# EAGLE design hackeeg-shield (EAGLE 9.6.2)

## Sheet 1 of 4: ADS1299 and power supplies
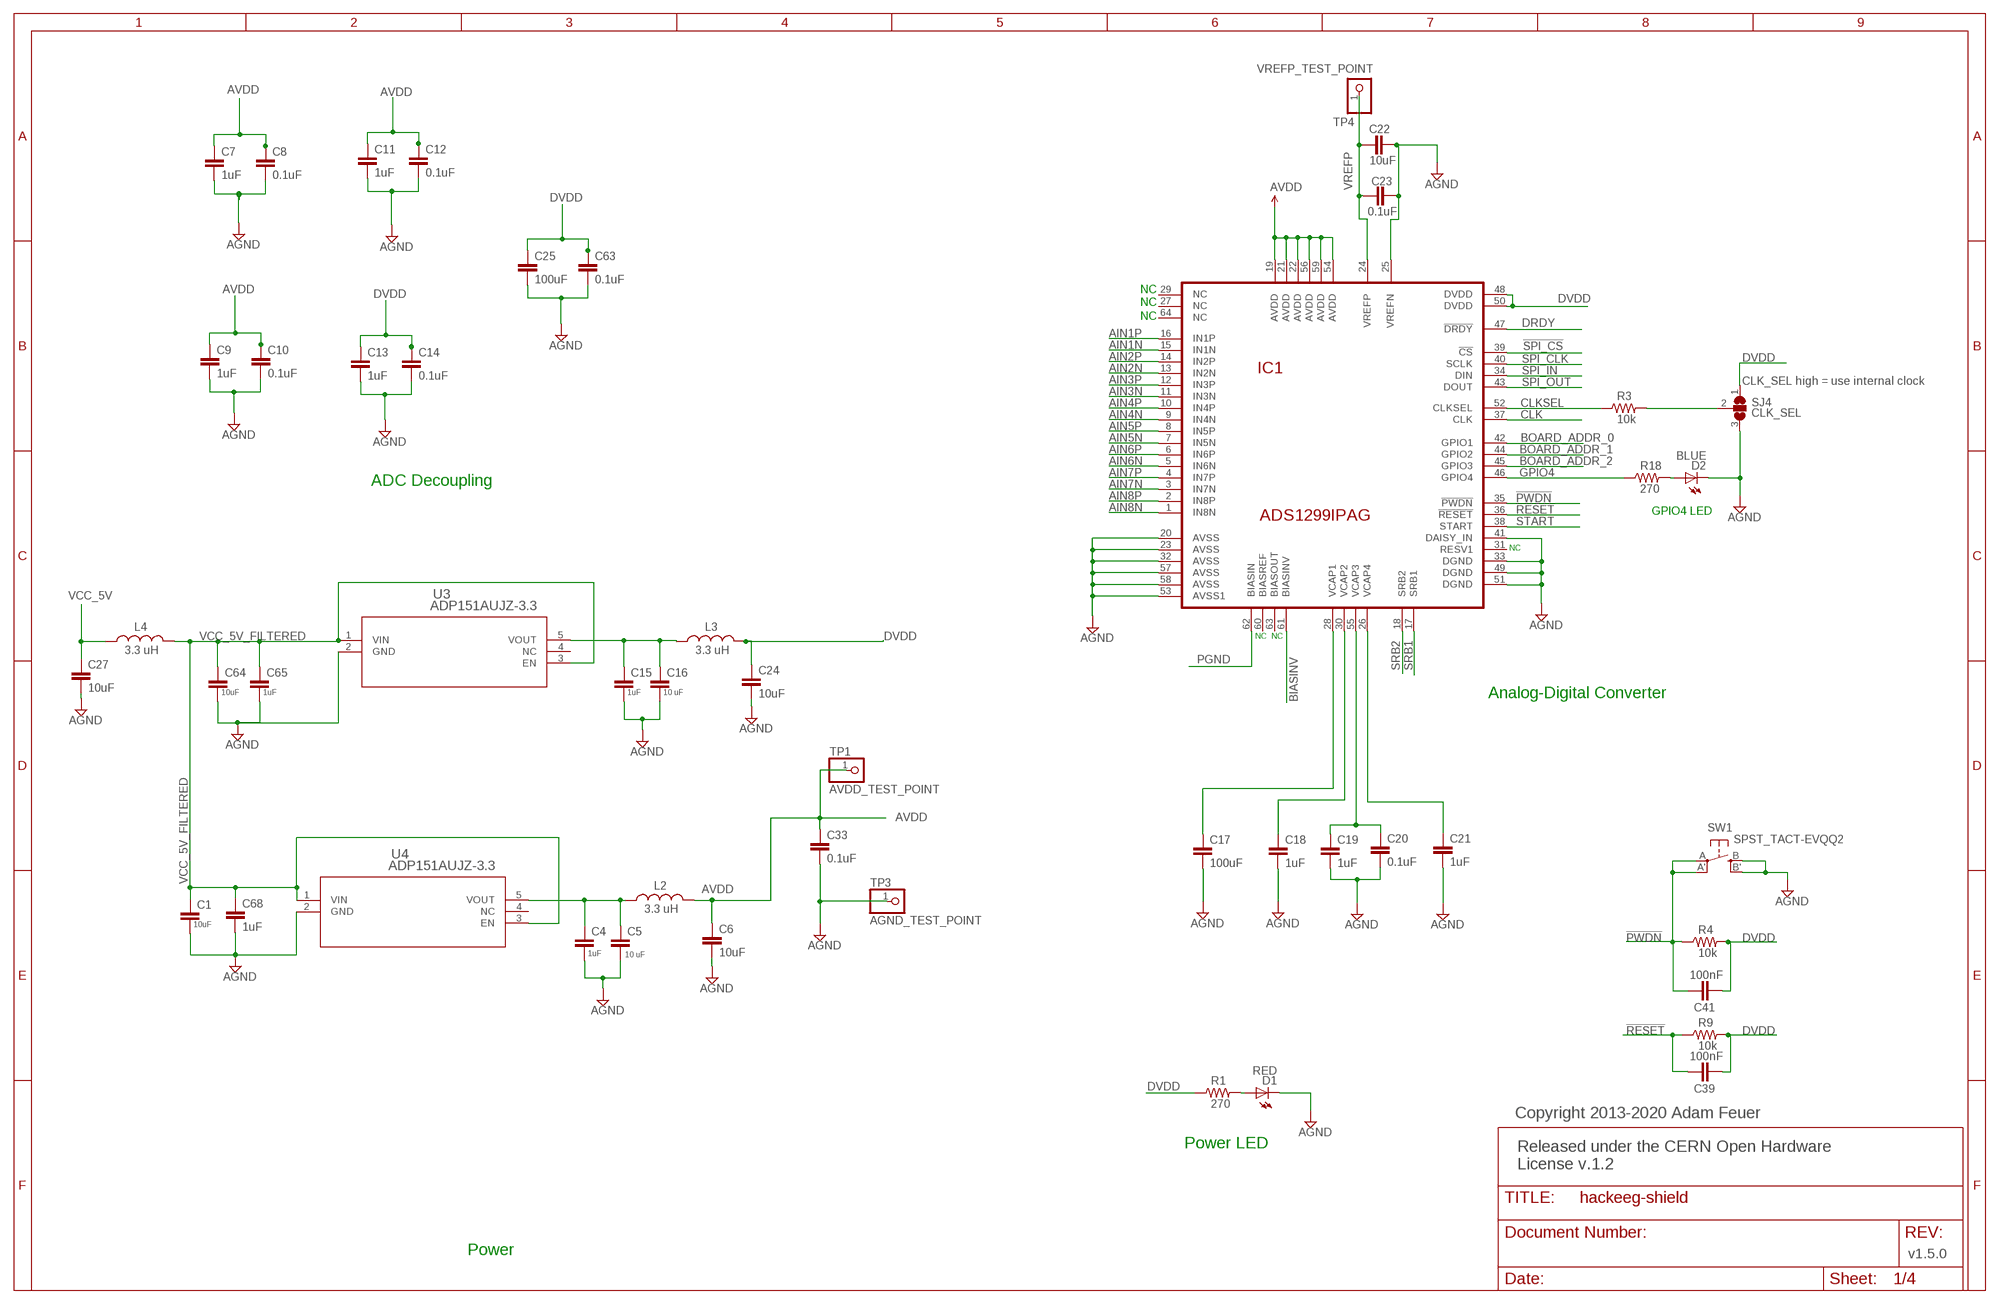
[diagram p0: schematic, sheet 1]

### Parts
C1  10uF  CAP0603-CAP  [0603-CAP]
C4  1uF  CAP0603-CAP  [0603-CAP]
C5  10 uF  CAP0603-CAP  [0603-CAP]
C6  10uF  CAP0603-CAP  [0603-CAP]
C7  1uF  CAP0603-CAP  [0603-CAP]
C8  0.1uF  CAP0603-CAP  [0603-CAP]
C9  1uF  CAP0603-CAP  [0603-CAP]
C10  0.1uF  CAP0603-CAP  [0603-CAP]
C11  1uF  CAP0603-CAP  [0603-CAP]
C12  0.1uF  CAP0603-CAP  [0603-CAP]
C13  1uF  CAP0603-CAP  [0603-CAP]
C14  0.1uF  CAP0603-CAP  [0603-CAP]
C15  1uF  CAP0603-CAP  [0603-CAP]
C16  10 uF  CAP0603-CAP  [0603-CAP]
C17  100uF  CAP1210  [1210]
C18  1uF  CAP0603-CAP  [0603-CAP]
C19  1uF  CAP0603-CAP  [0603-CAP]
C20  0.1uF  CAP0603-CAP  [0603-CAP]
C21  1uF  CAP0603-CAP  [0603-CAP]
C22  10uF  CAP0603-CAP  [0603-CAP]
C23  0.1uF  CAP0603-CAP  [0603-CAP]
C24  10uF  CAP0603-CAP  [0603-CAP]
C25  100uF  CAP1210  [1210]
C27  10uF  CAP0603-CAP  [0603-CAP]
C33  0.1uF  CAP0603-CAP  [0603-CAP]
C39  100nF  CAP0603-CAP  [0603-CAP]
C41  100nF  CAP0603-CAP  [0603-CAP]
C63  0.1uF  CAP0603-CAP  [0603-CAP]
C64  10uF  CAP0603-CAP  [0603-CAP]
C65  1uF  CAP0603-CAP  [0603-CAP]
C68  1uF  CAP0603-CAP  [0603-CAP]
D1  RED  LED-RED1206  [LED-1206]
D2  BLUE  LED-WHITE  [LED-1206]
IC1  ADS1299IPAG  ADS1299*PAG*  [TQFP64]
L2  3.3 uH  INDUCTOR0805  [0805]
L3  3.3 uH  INDUCTOR0805  [0805]
L4  3.3 uH  INDUCTOR0805  [0805]
R1  270  RESISTOR0603-RES  [0603-RES]
R3  10k  RESISTOR0603-RES  [0603-RES]
R4  10k  RESISTOR0603-RES  [0603-RES]
R9  10k  RESISTOR0603-RES  [0603-RES]
R18  270  RESISTOR0603-RES  [0603-RES]
SJ4  CLK_SEL  SJ2W  [SJ_2]
SW1  SPST_TACT-EVQQ2  [EVQ-Q2]
TP1  AVDD_TEST_POINT  PINHD-1X1  [1X01]
TP3  AGND_TEST_POINT  PINHD-1X1  [1X01]
TP4  VREFP_TEST_POINT  PINHD-1X1  [1X01]
U3  ADP151AUJZ-3.3  [UJ_5_ADI]
U4  ADP151AUJZ-3.3  [UJ_5_ADI]

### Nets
!PWDN: C41.1 IC1.35(!PWDN) R4.1 SW1.A'(P1) SW1.A(P)
!RESET: C39.1 IC1.36(!RESET) R9.1
!SPI_CS: IC1.39(!CS) ; also sheet 3
AGND: C1.2 C4.2 C5.2 C6.2 C7.2 C8.2 C9.2 C10.2 C11.2 C12.2 C13.2 C14.2 C15.2 C16.2 C17.2 C18.2 C19.2 C20.2 C21.2 C22.2 C23.2 C24.2 C25.2 C27.2 C33.2 C63.2 C64.2 C65.2 C68.2 D1.C D2.C IC1.20(AVSS) IC1.23(AVSS) IC1.25(VREFN) IC1.32(AVSS) IC1.33(DGND) IC1.41(DAISY_IN) IC1.49(DGND) IC1.51(DGND) IC1.53(AVSS1) IC1.57(AVSS) IC1.58(AVSS) SJ4.3 SW1.B'(S1) SW1.B(S) TP3.1 U3.2(GND) U4.2(GND) ; also sheet 2,3
AIN1N: IC1.15(IN1N) ; also sheet 2
AIN1P: IC1.16(IN1P) ; also sheet 2
AIN2N: IC1.13(IN2N) ; also sheet 2
AIN2P: IC1.14(IN2P) ; also sheet 2
AIN3N: IC1.11(IN3N) ; also sheet 2
AIN3P: IC1.12(IN3P) ; also sheet 2
AIN4N: IC1.9(IN4N) ; also sheet 2
AIN4P: IC1.10(IN4P) ; also sheet 2
AIN5N: IC1.7(IN5N) ; also sheet 2
AIN5P: IC1.8(IN5P) ; also sheet 2
AIN6N: IC1.5(IN6N) ; also sheet 2
AIN6P: IC1.6(IN6P) ; also sheet 2
AIN7N: IC1.3(IN7N) ; also sheet 2
AIN7P: IC1.4(IN7P) ; also sheet 2
AIN8N: IC1.1(IN8N) ; also sheet 2
AIN8P: IC1.2(IN8P) ; also sheet 2
AVDD: C6.1 C7.1 C8.1 C9.1 C10.1 C11.1 C12.1 C33.1 IC1.19(AVDD) IC1.21(AVDD) IC1.22(AVDD) IC1.54(AVDD) IC1.56(AVDD) IC1.59(AVDD) L2.2 TP1.1 ; also sheet 2
BIASINV: IC1.61(BIASINV) ; also sheet 2
BOARD_ADDR_0: IC1.42(GPIO1)
BOARD_ADDR_1: IC1.44(GPIO2)
BOARD_ADDR_2: IC1.45(GPIO3)
CLK: IC1.37(CLK) ; also sheet 3
CLKSEL: IC1.52(CLKSEL) R3.1
DRDY: IC1.47(!DRDY) ; also sheet 3
DVDD: C13.1 C14.1 C24.1 C25.1 C39.2 C41.2 C63.1 IC1.48(DVDD) IC1.50(DVDD) L3.2 R1.1 R4.2 R9.2 SJ4.1 ; also sheet 3
GPIO4: IC1.46(GPIO4) R18.1
N$1: C4.1 C5.1 L2.1 U4.5(VOUT)
N$2: C15.1 C16.1 L3.1 U3.5(VOUT)
N$3: C17.1 IC1.28(VCAP1)
N$4: C18.1 IC1.30(VCAP2)
N$5: C19.1 C20.1 IC1.55(VCAP3)
N$8: C21.1 IC1.26(VCAP4)
N$14: D2.A R18.2
N$19: D1.A R1.2
N$20: R3.2 SJ4.2
PGND: IC1.62(BIASIN) ; also sheet 2
SPI_CLK: IC1.40(SCLK) ; also sheet 3
SPI_IN: IC1.34(DIN) ; also sheet 3
SPI_OUT: IC1.43(DOUT) ; also sheet 3
SRB1: IC1.17(SRB1) ; also sheet 2
SRB2: IC1.18(SRB2) ; also sheet 3
START: IC1.38(START) ; also sheet 3
VCC_5V: C27.1 L4.1 ; also sheet 3
VCC_5V_FILTERED: C1.1 C64.1 C65.1 C68.1 L4.2 U3.1(VIN) U3.3(EN) U4.1(VIN) U4.3(EN)
VREFP: C22.1 C23.1 IC1.24(VREFP) TP4.1
Unconnected: IC1.27(NC) IC1.29(NC) IC1.31(RESV1) IC1.60(BIASREF) IC1.63(BIASOUT) IC1.64(NC) U3.4(NC) U4.4(NC)

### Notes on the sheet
- NC
- NC
- NC
- CLK_SEL high = use internal clock
- ADC Decoupling
- GPIO4 LED
- NC
- NC | NC
- Analog-Digital Converter
- Copyright 2013-2020 Adam Feuer
- Power LED
- Released under the CERN Open Hardware 
  License v.1.2
- Power | v1.5.0

## Sheet 2 of 4: Input filtering and electrode connector
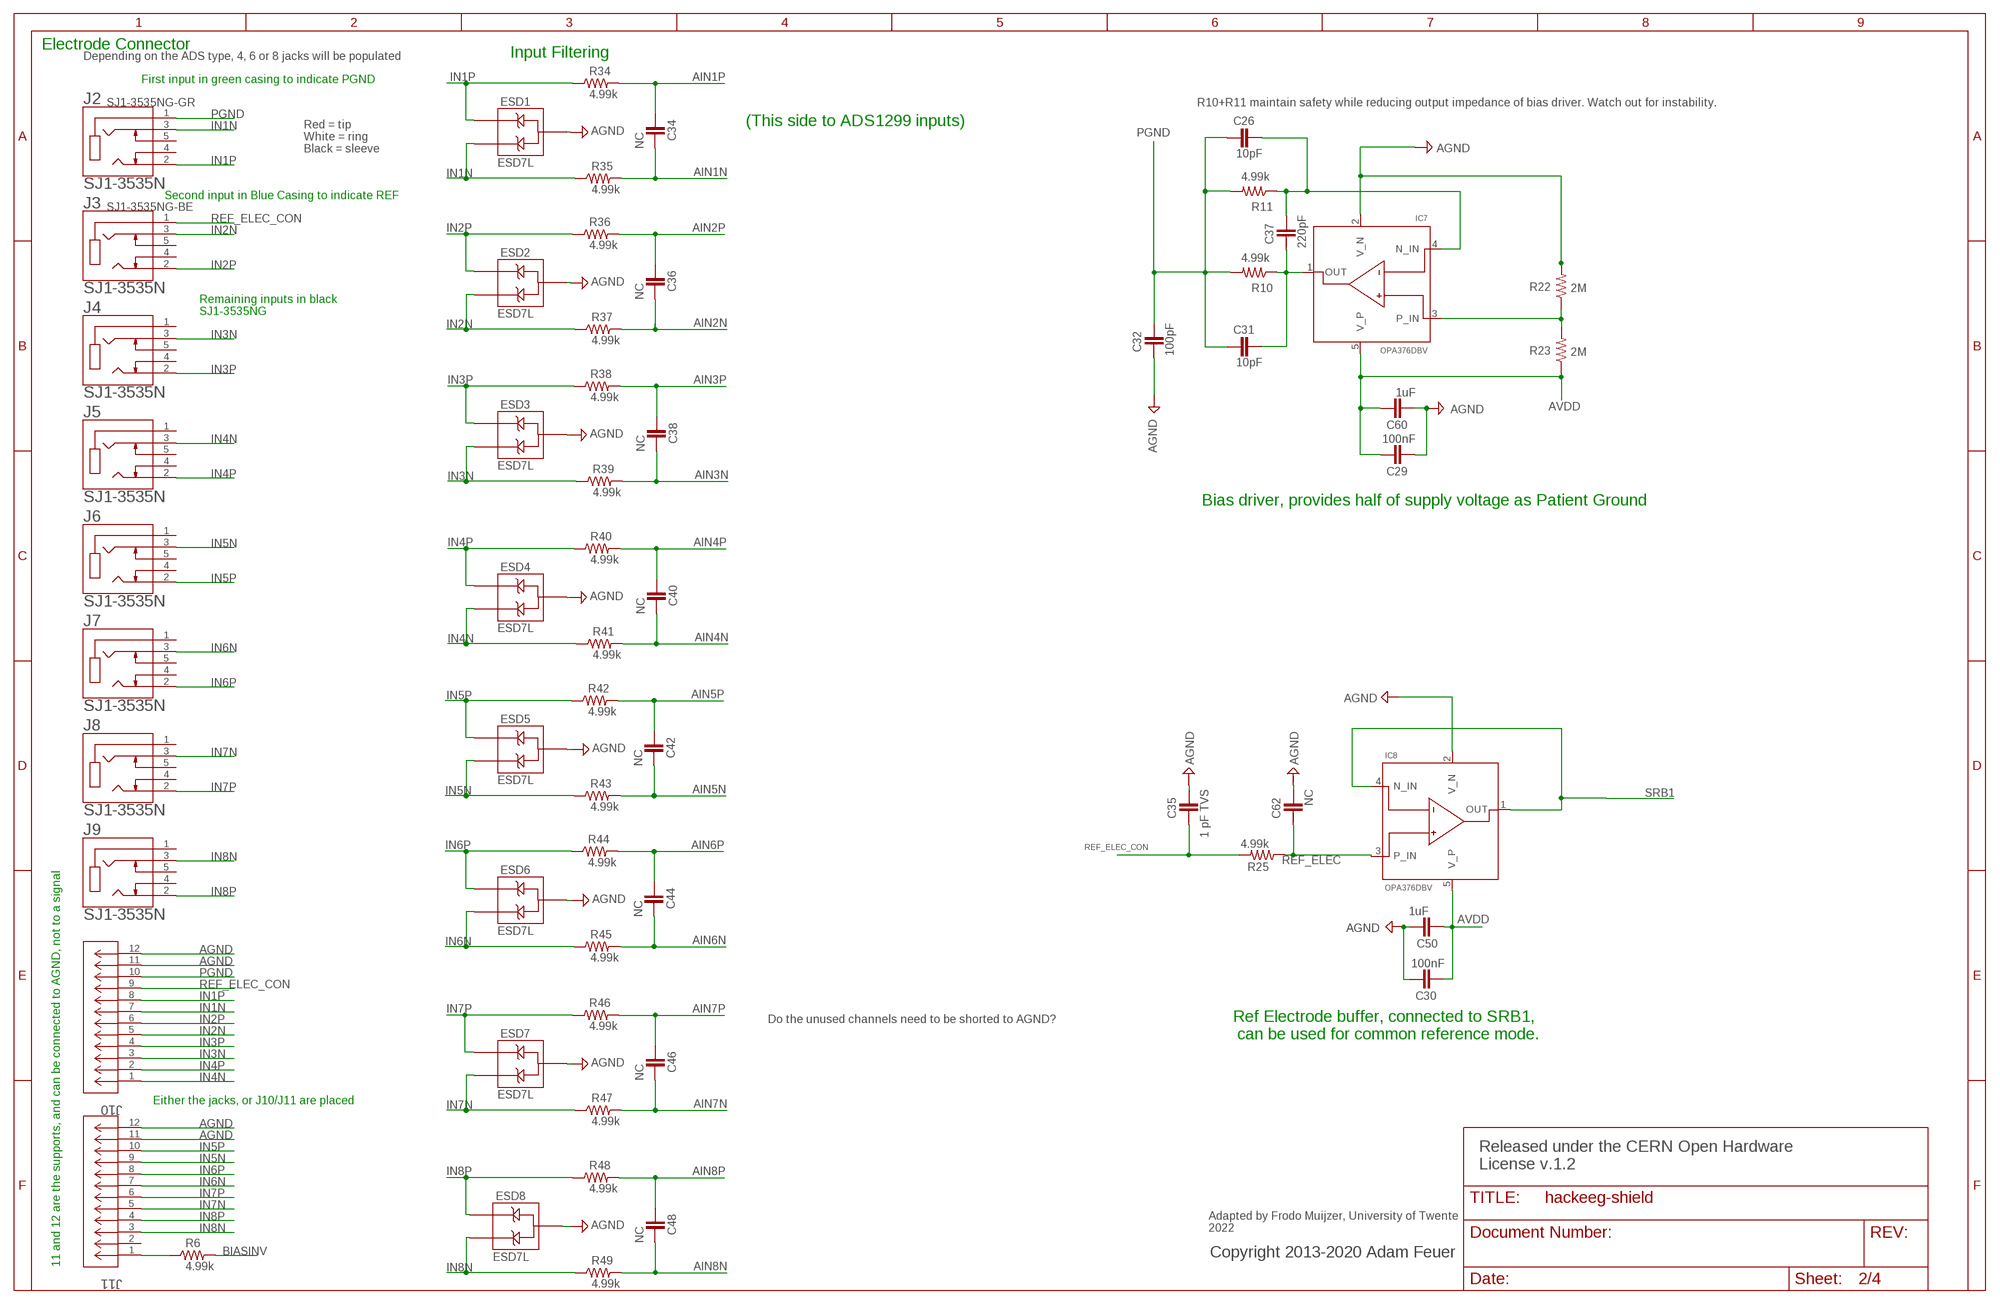
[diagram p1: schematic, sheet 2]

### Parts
C26  10pF  CAP0603-CAP  [0603-CAP]
C29  100nF  CAP0603-CAP  [0603-CAP]
C30  100nF  CAP0603-CAP  [0603-CAP]
C31  10pF  CAP0603-CAP  [0603-CAP]
C32  100pF  CAP0603-CAP  [0603-CAP]
C34  NC  CAP0603-CAP  [0603-CAP]
C35  1 pF TVS  CAP0603-CAP  [0603-CAP]
C36  NC  CAP0603-CAP  [0603-CAP]
C37  220pF  CAP0603-CAP  [0603-CAP]
C38  NC  CAP0603-CAP  [0603-CAP]
C40  NC  CAP0603-CAP  [0603-CAP]
C42  NC  CAP0603-CAP  [0603-CAP]
C44  NC  CAP0603-CAP  [0603-CAP]
C46  NC  CAP0603-CAP  [0603-CAP]
C48  NC  CAP0603-CAP  [0603-CAP]
C50  1uF  CAP0603-CAP  [0603-CAP]
C60  1uF  CAP0603-CAP  [0603-CAP]
C62  NC  CAP0603-CAP  [0603-CAP]
ESD1  ESD7L  [SOT-723]
ESD2  ESD7L  [SOT-723]
ESD3  ESD7L  [SOT-723]
ESD4  ESD7L  [SOT-723]
ESD5  ESD7L  [SOT-723]
ESD6  ESD7L  [SOT-723]
ESD7  ESD7L  [SOT-723]
ESD8  ESD7L  [SOT-723]
IC7  OPA376DBV  [SOT23-5]
IC8  OPA376DBV  [SOT23-5]
J2  SJ1-3535N  [CUI_SJ1-3535N]
J3  SJ1-3535N  [CUI_SJ1-3535N]
J4  SJ1-3535N  [CUI_SJ1-3535N]
J5  SJ1-3535N  [CUI_SJ1-3535N]
J6  SJ1-3535N  [CUI_SJ1-3535N]
J7  SJ1-3535N  [CUI_SJ1-3535N]
J8  SJ1-3535N  [CUI_SJ1-3535N]
J9  SJ1-3535N  [CUI_SJ1-3535N]
J10  533981071  [CON_533981071]
J11  533981071  [CON_533981071]
R6  4.99k  RESISTOR0603-RES  [0603-RES]
R10  4.99k  RESISTOR0603-RES  [0603-RES]
R11  4.99k  RESISTOR0603-RES  [0603-RES]
R22  2M  RESISTOR0603-RES  [0603-RES]
R23  2M  RESISTOR0603-RES  [0603-RES]
R25  4.99k  RESISTOR0603-RES  [0603-RES]
R34  4.99k  RESISTOR0603-RES  [0603-RES]
R35  4.99k  RESISTOR0603-RES  [0603-RES]
R36  4.99k  RESISTOR0603-RES  [0603-RES]
R37  4.99k  RESISTOR0603-RES  [0603-RES]
R38  4.99k  RESISTOR0603-RES  [0603-RES]
R39  4.99k  RESISTOR0603-RES  [0603-RES]
R40  4.99k  RESISTOR0603-RES  [0603-RES]
R41  4.99k  RESISTOR0603-RES  [0603-RES]
R42  4.99k  RESISTOR0603-RES  [0603-RES]
R43  4.99k  RESISTOR0603-RES  [0603-RES]
R44  4.99k  RESISTOR0603-RES  [0603-RES]
R45  4.99k  RESISTOR0603-RES  [0603-RES]
R46  4.99k  RESISTOR0603-RES  [0603-RES]
R47  4.99k  RESISTOR0603-RES  [0603-RES]
R48  4.99k  RESISTOR0603-RES  [0603-RES]
R49  4.99k  RESISTOR0603-RES  [0603-RES]

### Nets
AGND: C29.2 C30.1 C32.1 C35.2 C50.2 C60.2 C62.2 ESD1.P$3 ESD2.P$3 ESD3.P$3 ESD4.P$3 ESD5.P$3 ESD6.P$3 ESD7.P$3 ESD8.P$3 IC7.2(V_N) IC8.2(V_N) J10.11 J10.12 J11.11 J11.12 R22.2 ; also sheet 1,3
AIN1N: C34.2 R35.2 ; also sheet 1
AIN1P: C34.1 R34.2 ; also sheet 1
AIN2N: C36.2 R37.2 ; also sheet 1
AIN2P: C36.1 R36.2 ; also sheet 1
AIN3N: C38.2 R39.2 ; also sheet 1
AIN3P: C38.1 R38.2 ; also sheet 1
AIN4N: C40.2 R41.2 ; also sheet 1
AIN4P: C40.1 R40.2 ; also sheet 1
AIN5N: C42.2 R43.2 ; also sheet 1
AIN5P: C42.1 R42.2 ; also sheet 1
AIN6N: C44.2 R45.2 ; also sheet 1
AIN6P: C44.1 R44.2 ; also sheet 1
AIN7N: C46.2 R47.2 ; also sheet 1
AIN7P: C46.1 R46.2 ; also sheet 1
AIN8N: C48.2 R49.2 ; also sheet 1
AIN8P: C48.1 R48.2 ; also sheet 1
AVDD: C29.1 C30.2 C50.1 C60.1 IC7.5(V_P) IC8.5(V_P) R23.1 ; also sheet 1
BIASINV: R6.2 ; also sheet 1
IN1N: ESD1.P$2 J2.3 J10.7 R35.1
IN1P: ESD1.P$1 J2.2 J10.8 R34.1
IN2N: ESD2.P$2 J3.3 J10.5 R37.1
IN2P: ESD2.P$1 J3.2 J10.6 R36.1
IN3N: ESD3.P$2 J4.3 J10.3 R39.1
IN3P: ESD3.P$1 J4.2 J10.4 R38.1
IN4N: ESD4.P$2 J5.3 J10.1 R41.1
IN4P: ESD4.P$1 J5.2 J10.2 R40.1
IN5N: ESD5.P$2 J6.3 J11.9 R43.1
IN5P: ESD5.P$1 J6.2 J11.10 R42.1
IN6N: ESD6.P$2 J7.3 J11.7 R45.1
IN6P: ESD6.P$1 J7.2 J11.8 R44.1
IN7N: ESD7.P$2 J8.3 J11.5 R47.1
IN7P: ESD7.P$1 J8.2 J11.6 R46.1
IN8N: ESD8.P$2 J9.3 J11.3 R49.1
IN8P: ESD8.P$1 J9.2 J11.4 R48.1
N$10: J11.1 R6.1
N$15: IC7.3(P_IN) R22.1 R23.2
N$18: C31.2 C37.1 IC7.1(OUT) R10.1
N$54: C26.2 C37.2 IC7.4(N_IN) R11.1
PGND: C26.1 C31.1 C32.2 J2.1 J10.10 R10.2 R11.2 ; also sheet 1
REF_ELEC: C62.1 IC8.3(P_IN) R25.1
REF_ELEC_CON: C35.1 J3.1 J10.9 R25.2
SRB1: IC8.1(OUT) IC8.4(N_IN) ; also sheet 1
Unconnected: J2.4 J2.5 J3.4 J3.5 J4.1 J4.4 J4.5 J5.1 J5.4 J5.5 J6.1 J6.4 J6.5 J7.1 J7.4 J7.5 J8.1 J8.4 J8.5 J9.1 J9.4 J9.5 J11.2

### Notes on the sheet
- Electrode Connector
- Depending on the ADS type, 4, 6 or 8 jacks will be populated | Input Filtering
- First input in green casing to indicate PGND
- R10+R11 maintain safety while reducing output impedance of bias driver. Watch out for instability.
- (This side to ADS1299 inputs)
- Red = tip
  White = ring
  Black = sleeve
- Second input in Blue Casing to indicate REF
- Remaining inputs in black
  SJ1-3535NG
- Bias driver, provides half of supply voltage as Patient Ground
- Do the unused channels need to be shorted to AGND?
- Ref Electrode buffer, connected to SRB1,
   can be used for common reference mode.
- Either the jacks, or J10/J11 are placed
- Released under the CERN Open Hardware 
  License v.1.2
- Adapted by Frodo Muijzer, University of Twente
  2022
- Copyright 2013-2020 Adam Feuer
- 11 and 12 are the supports, and can be connected to AGND, not to a signal

## Sheet 3 of 4: Board to board connectors, isolation and additional connector.
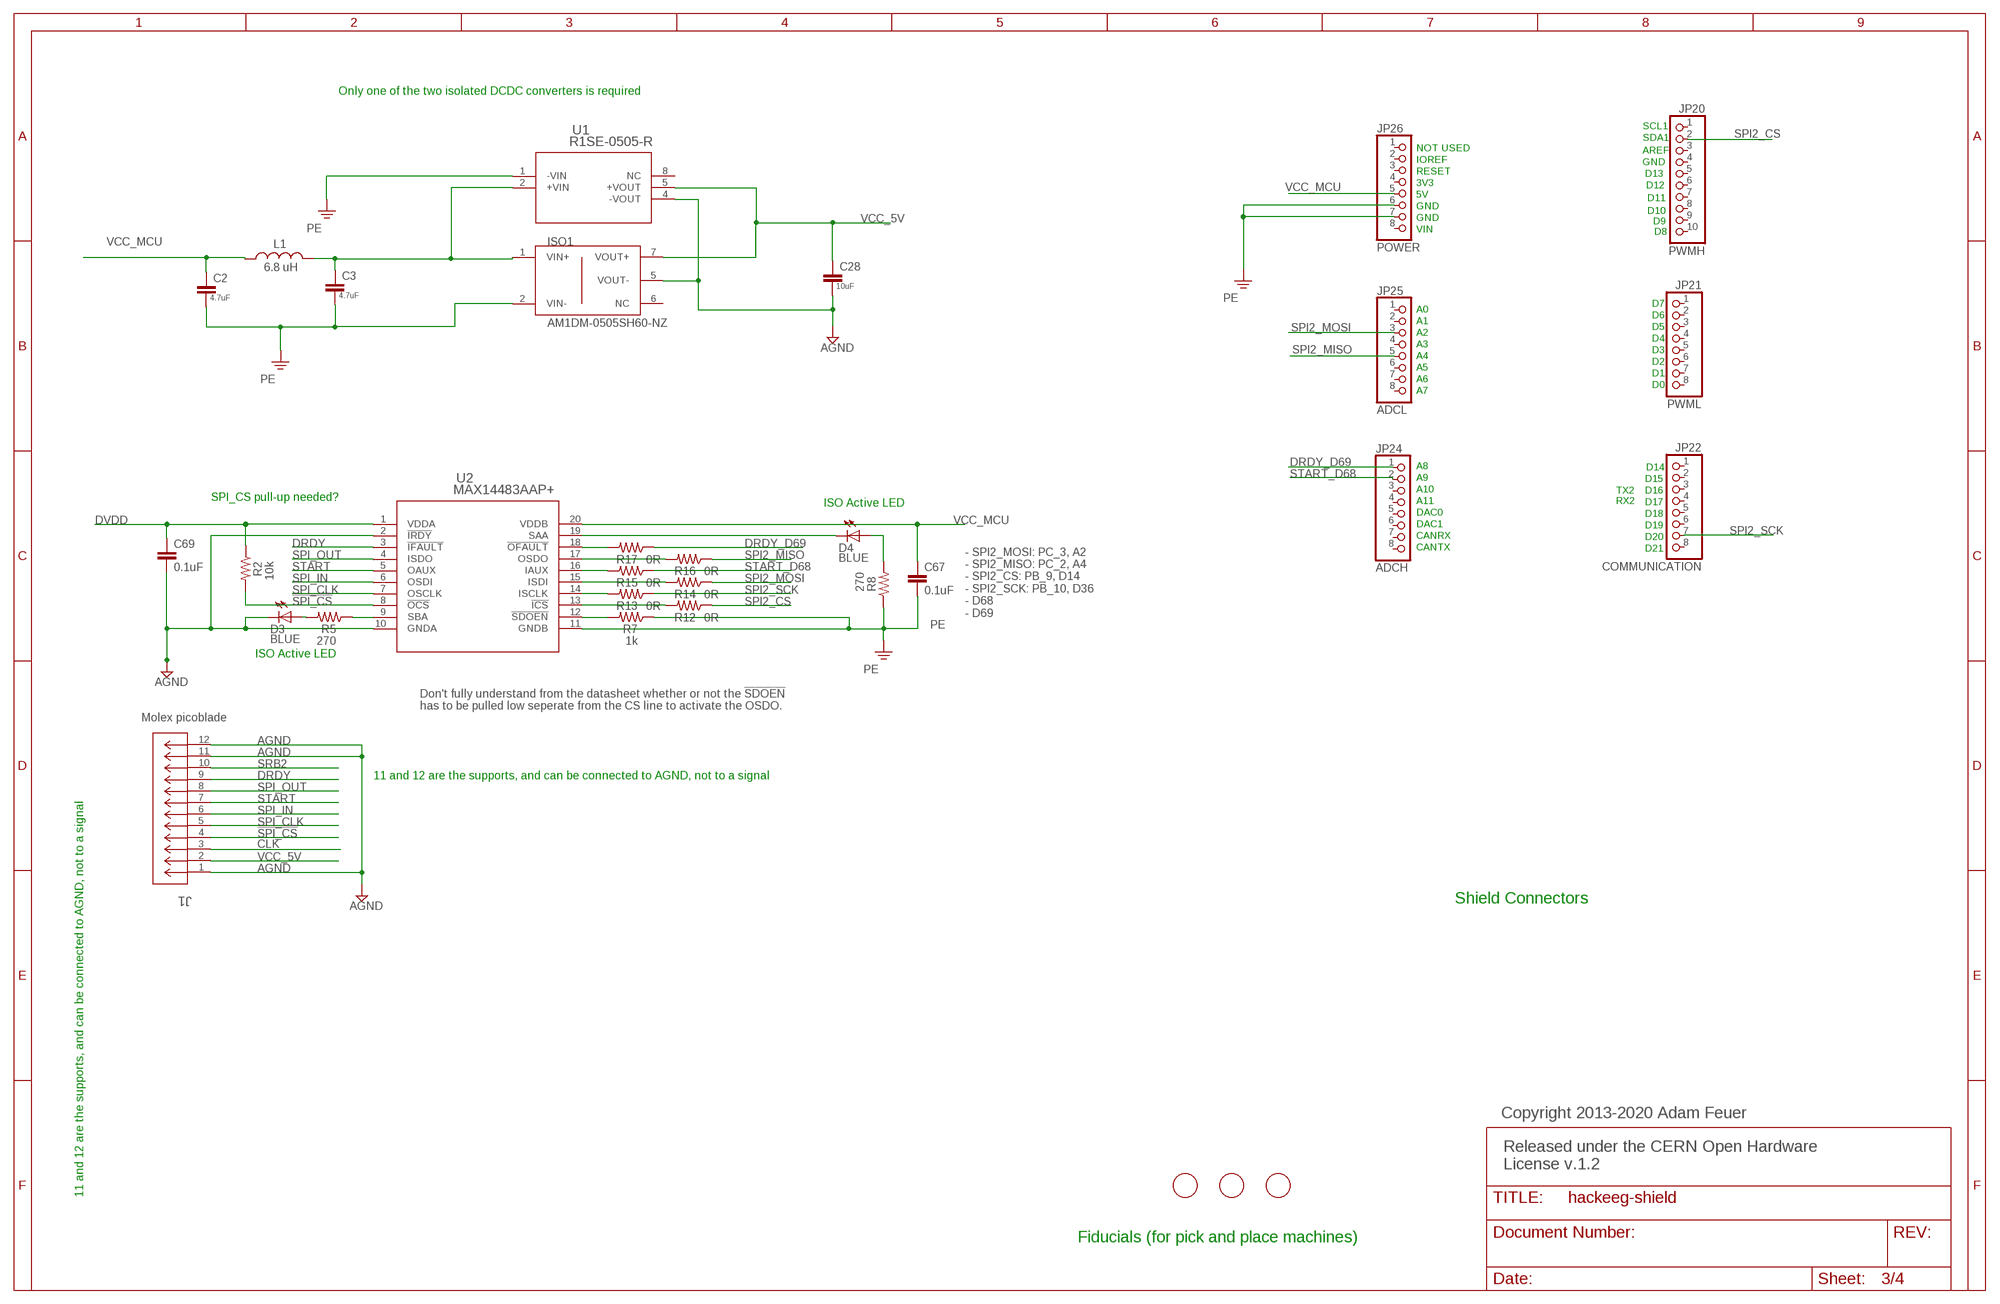
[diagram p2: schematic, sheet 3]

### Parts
C2  4.7uF  CAP0603-CAP  [0603-CAP]
C3  4.7uF  CAP0603-CAP  [0603-CAP]
C28  10uF  CAP0603-CAP  [0603-CAP]
C67  0.1uF  CAP0603-CAP  [0603-CAP]
C69  0.1uF  CAP0603-CAP  [0603-CAP]
D3  BLUE  LED-WHITE  [LED-1206]
D4  BLUE  LED-WHITE  [LED-1206]
ISO1  AM1DM-0505SH60-NZ  [SIP1005W50P254L1965H1265Q7]
J1  533981071  [CON_533981071]
JP20  PWMH  PINHD-1X10  [1X10]
JP21  PWML  PINHD-1X8  [1X08]
JP22  COMMUNICATION  PINHD-1X8  [1X08]
JP24  ADCH  PINHD-1X8  [1X08]
JP25  ADCL  PINHD-1X8  [1X08]
JP26  POWER  PINHD-1X8  [1X08]
L1  6.8 uH  INDUCTOR0805  [0805]
R2  10k  RESISTOR0603-RES  [0603-RES]
R5  270  RESISTOR0603-RES  [0603-RES]
R7  1k  RESISTOR0603-RES  [0603-RES]
R8  270  RESISTOR0603-RES  [0603-RES]
R12  0R  RESISTOR0603-RES  [0603-RES]
R13  0R  RESISTOR0603-RES  [0603-RES]
R14  0R  RESISTOR0603-RES  [0603-RES]
R15  0R  RESISTOR0603-RES  [0603-RES]
R16  0R  RESISTOR0603-RES  [0603-RES]
R17  0R  RESISTOR0603-RES  [0603-RES]
U1  R1SE-0505-R  [R1SE-0505-R_RCP]
U2  MAX14483AAP+  [21-0056C_20_MXM]
U$2  FIDUCIAL  [FIDUCIAL_1MM]
U$5  FIDUCIAL  [FIDUCIAL_1MM]
U$6  FIDUCIAL  [FIDUCIAL_1MM]

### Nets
!SPI_CS: J1.4 R2.2 U2.8(!OCS) ; also sheet 1
AGND: C28.2 C69.2 D3.C ISO1.5(VOUT-) J1.1 J1.11 J1.12 U1.4(-VOUT) U2.2(!IRDY) U2.10(GNDA) ; also sheet 1,2
CLK: J1.3 ; also sheet 1
DRDY: J1.9 U2.3(!IFAULT) ; also sheet 1
DRDY_D69: JP24.1 R17.1
DVDD: C69.1 R2.1 U2.1(VDDA) ; also sheet 1
N$6: C3.1 ISO1.1(VIN+) L1.2 U1.2(+VIN)
N$7: D4.A R8.2
N$9: D3.A R5.2
N$11: R5.1 U2.9(SBA)
N$12: R17.2 U2.18(!OFAULT)
N$13: D4.C U2.19(SAA)
N$16: R12.2 U2.13(!ICS)
N$17: R13.2 U2.14(ISCLK)
N$21: R14.2 U2.15(ISDI)
N$22: R15.2 U2.16(IAUX)
N$23: R16.2 U2.17(OSDO)
N$44: R7.2 U2.12(!SDOEN)
PE: C2.2 C3.2 C67.2 ISO1.2(VIN-) JP26.6 JP26.7 R7.1 R8.1 U1.1(-VIN) U2.11(GNDB)
SPI2_CS: JP20.2 R12.1
SPI2_MISO: JP25.5 R16.1
SPI2_MOSI: JP25.3 R14.1
SPI2_SCK: JP22.7 R13.1
SPI_CLK: J1.5 U2.7(OSCLK) ; also sheet 1
SPI_IN: J1.6 U2.6(OSDI) ; also sheet 1
SPI_OUT: J1.8 U2.4(ISDO) ; also sheet 1
SRB2: J1.10 ; also sheet 1
START: J1.7 U2.5(OAUX) ; also sheet 1
START_D68: JP24.2 R15.1
VCC_5V: C28.1 ISO1.7(VOUT+) J1.2 U1.5(+VOUT) ; also sheet 1
VCC_MCU: C2.1 C67.1 JP26.5 L1.1 U2.20(VDDB)
Unconnected: ISO1.6(NC) JP20.1 JP20.3 JP20.4 JP20.5 JP20.6 JP20.7 JP20.8 JP20.9 JP20.10 JP21.1 JP21.2 JP21.3 JP21.4 JP21.5 JP21.6 JP21.7 JP21.8 JP22.1 JP22.2 JP22.3 JP22.4 JP22.5 JP22.6 JP22.8 JP24.3 JP24.4 JP24.5 JP24.6 JP24.7 JP24.8 JP25.1 JP25.2 JP25.4 JP25.6 JP25.7 JP25.8 JP26.1 JP26.2 JP26.3 JP26.4 JP26.8 U1.8(NC)

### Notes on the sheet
- Only one of the two isolated DCDC converters is required
- SCL1
- SDA1
- NOT USED | AREF
- IOREF | GND
- RESET | D13
- 3V3 | D12
- 5V
- D11
- GND
- D10
- GND
- D9
- VIN | D8
- D7
- A0
- D6
- A1
- D5
- A2
- D4
- A3
- D3
- A4
- D2
- A5
- D1
- A6
- D0
- A7
- A8 | D14
- A9 | D15
- A10 | TX2 | D16
- SPI_CS pull-up needed? | ISO Active LED
- A11 | RX2 | D17
- DAC0 | D18
- DAC1 | D19
- CANRX | D20
- CANTX | D21
- - SPI2_MOSI: PC_3, A2 
  - SPI2_MISO: PC_2, A4 
  - SPI2_CS: PB_9, D14 
  - SPI2_SCK: PB_10, D36
  - D68
  - D69
- ISO Active LED
- Don't fully understand from the datasheet whether or not the !SDOEN
  has to be pulled low seperate from the CS line to activate the OSDO.
- Molex picoblade
- 11 and 12 are the supports, and can be connected to AGND, not to a signal
- Shield Connectors
- Copyright 2013-2020 Adam Feuer
- Released under the CERN Open Hardware 
  License v.1.2
- 11 and 12 are the supports, and can be connected to AGND, not to a signal
- Fiducials (for pick and place machines)

## Sheet 4 of 4: Nucleo headers
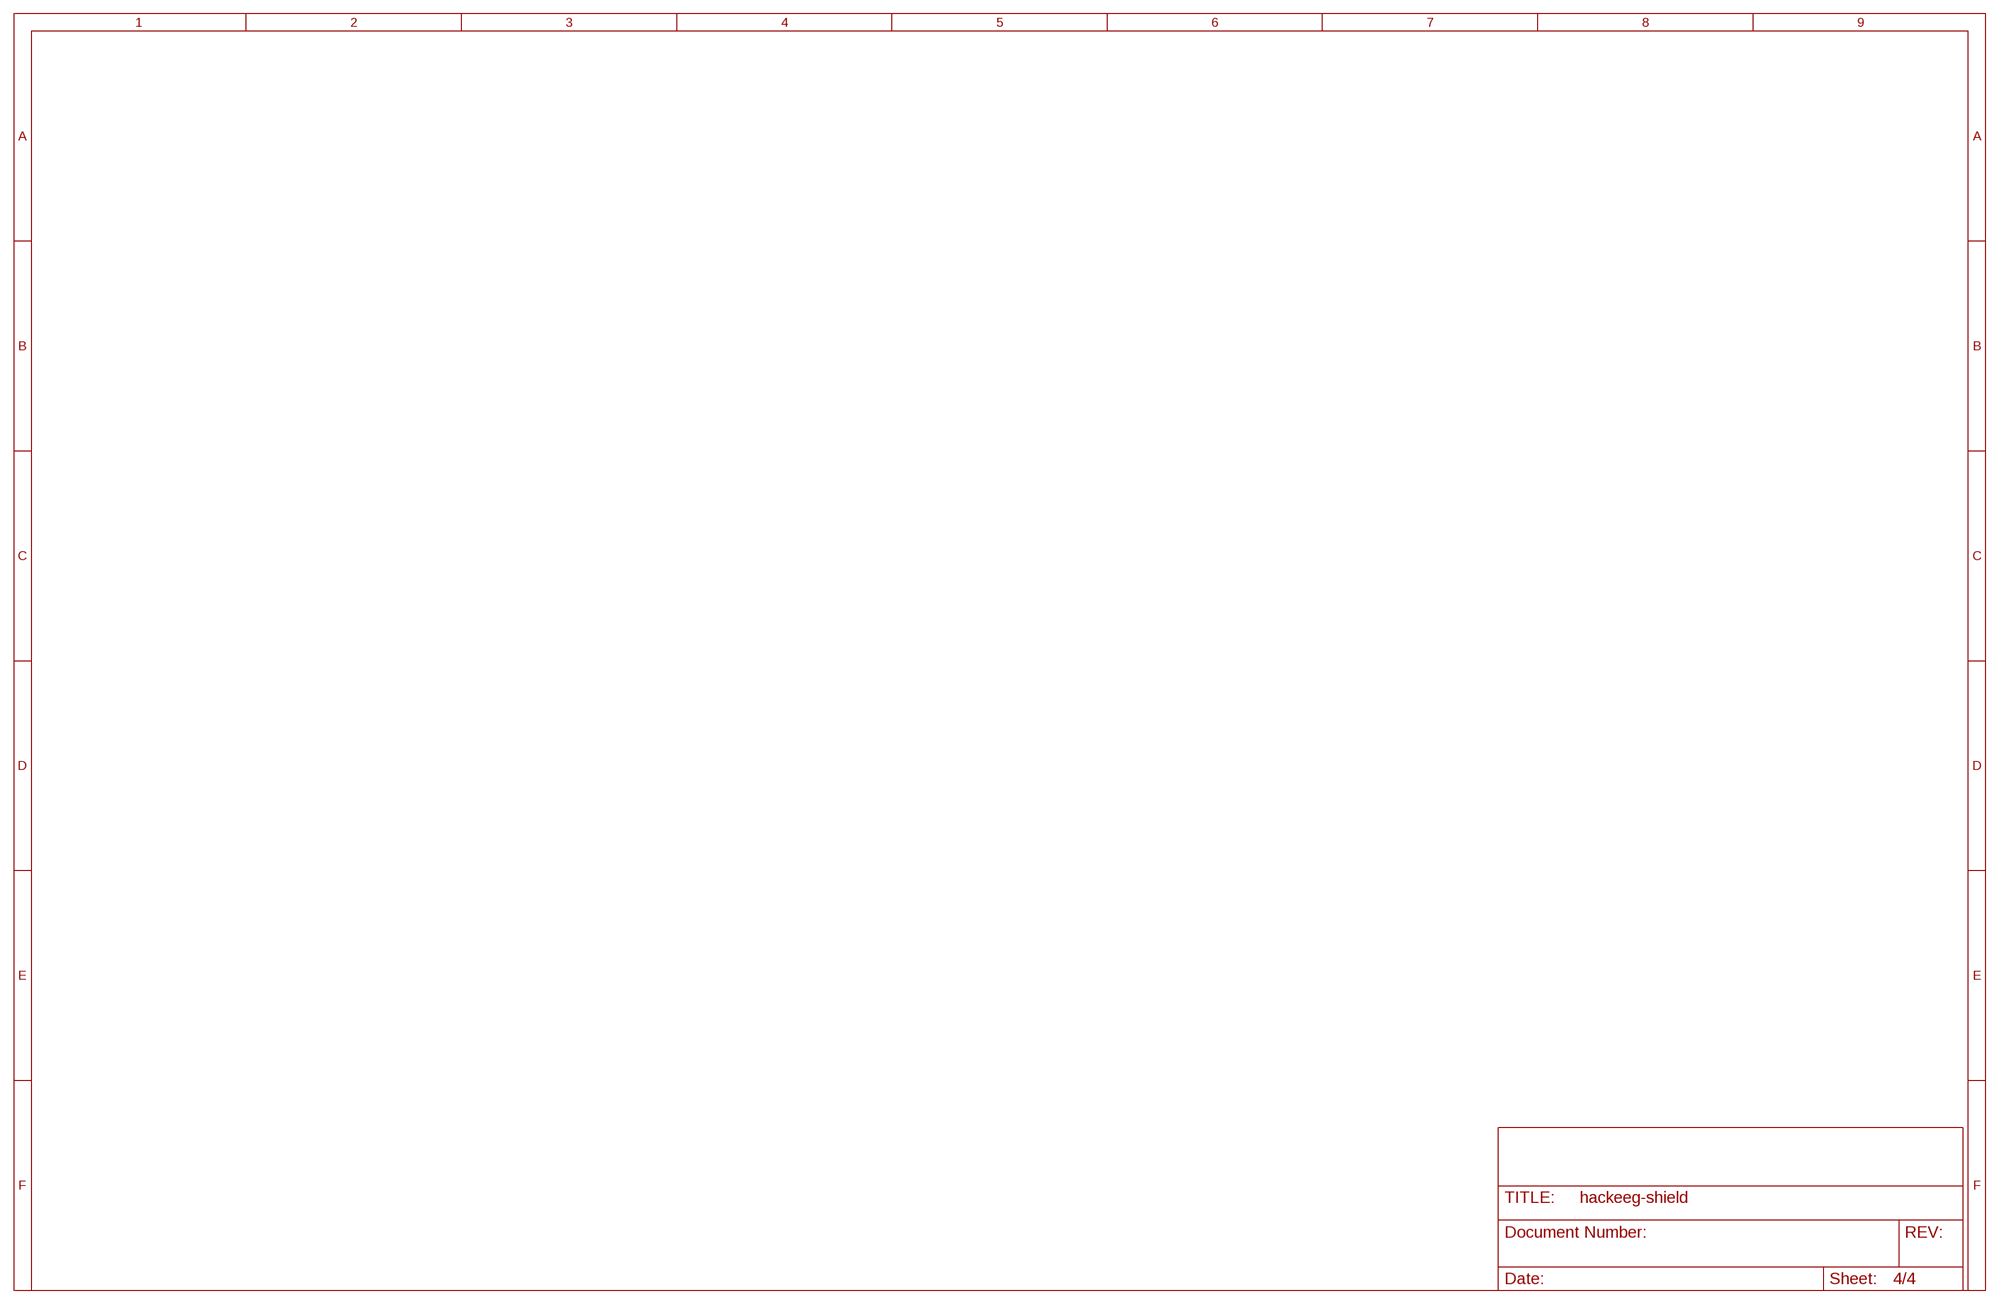
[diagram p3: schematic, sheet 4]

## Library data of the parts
C1-C42 C44 C46 C48 C50 C60 C62-C65 C67-C69 = SparkFun-Passives:CAP: Capacitor
D1 = SparkFun-LED:LED-RED: Assorted Red LEDs; PROD_ID: DIO-00809
D2-D4 = SparkFun-LED:LED-WHITE: White SMD LEDs; PROD_ID: DIO-09955; VALUE: WHITE
ESD1-ESD8 = ESD7L:ESD7L: PolMar Check availability; AVAILABILITY: In Stock; DESCRIPTION: 10.4V Clamp 1A (8/20µs) Ipp Tvs Diode Surface Mount SOT-723; MF: ON Semiconductor; MP: ESD7L; PACKAGE: SOT-723 ON Semiconductor; PRICE: None; PURCHASE-URL: https://pricing.snapeda.com/search/part/ESD7L/?ref=eda
IC1 = ADS129x:ADS1299: 8-Channel, 24-Bit Analog-To-Digital Converter With Integrated EEG Front End. ADS1299 modifications by Adam Feuer (adam@adamfeuer.com) Based on ADS1298: Drawn 23.07.2011 by Tomasz Boleslaw CEDRO (http://www.tomek.cedro.info).
IC7 IC8 = OPA376:OPA376: Low-Noise, Low Quiescent Current, Precision Operational Amplifier
ISO1 = Aimtec AM1D:AM1DM-0505SH60-NZ: AM1DM-0505SH60-NZ - FEATURES: • 7 pin SIP package • High efficiency up to 81% • Reinforced insulation • Leakage current 2µA • Operating temperature -40° C to + 85° C • Isolation voltage: 4200VAC or 6000VDC • Ultra-low Isolation capacitance of 5pF • IEC/EN/UL60601-1 • 1xMOPP/2xMOOP
J1 J10 J11 = Molex Picoblade 53398-1071:533981071; COPYRIGHT: Copyright (C) 2022 Ultra Librarian. All rights reserved.; MANUFACTURER_PART_NUMBER: 533981071; MFR_NAME: Molex Connector Corporation
J2 = SJ1-3535N:SJ1-3535N: SJ1 Series 3.5 mm 12 V Right Angle Through Hole Isolated Stereo Audio Jack Check availability; AVAILABILITY: In Stock; CUI_PURCHASE_URL: https://www.cuidevices.com/product/interconnect/connectors/audio-connectors/jacks/sj1-353xn-series?utm_source=snapeda.com&utm_medium=referral&utm_campaign=snapedaBOM; DESCRIPTION: 3.5 mm, Stereo, Right Angle, Through Hole, Audio Jack Connector; MF: CUI Devices; MP: SJ1-3535NG-GR; PACKAGE: None; PRICE: None; PURCHASE-URL: https://pricing.snapeda.com/search/part/SJ1-3535N/?ref=eda
J3 = SJ1-3535N:SJ1-3535N: SJ1 Series 3.5 mm 12 V Right Angle Through Hole Isolated Stereo Audio Jack Check availability; AVAILABILITY: In Stock; CUI_PURCHASE_URL: https://www.cuidevices.com/product/interconnect/connectors/audio-connectors/jacks/sj1-353xn-series?utm_source=snapeda.com&utm_medium=referral&utm_campaign=snapedaBOM; DESCRIPTION: 3.5 mm, Stereo, Right Angle, Through Hole, Audio Jack Connector; MF: CUI Devices; MP: SJ1-3535NG-BE; PACKAGE: None; PRICE: None; PURCHASE-URL: https://pricing.snapeda.com/search/part/SJ1-3535N/?ref=eda
J4-J9 = SJ1-3535N:SJ1-3535N: SJ1 Series 3.5 mm 12 V Right Angle Through Hole Isolated Stereo Audio Jack Check availability; AVAILABILITY: In Stock; CUI_PURCHASE_URL: https://www.cuidevices.com/product/interconnect/connectors/audio-connectors/jacks/sj1-353xn-series?utm_source=snapeda.com&utm_medium=referral&utm_campaign=snapedaBOM; DESCRIPTION: 3.5 mm, Stereo, Right Angle, Through Hole, Audio Jack Connector; MF: CUI Devices; MP: SJ1-3535N; PACKAGE: None; PRICE: None; PURCHASE-URL: https://pricing.snapeda.com/search/part/SJ1-3535N/?ref=eda
JP20 = SmartPrj:PINHD-1X10: PIN HEADER
JP21 JP22 JP24-JP26 = SmartPrj:PINHD-1X8: PIN HEADER
L1-L4 = SparkFun-Passives:INDUCTOR: Inductors
R1-R18 R22 R23 R25 R34-R49 = SparkFun-Passives:RESISTOR: Resistor
SJ4 = jumper:SJ2W: SMD solder JUMPER
SW1 = adafruit:SPST_TACT: SMT 6mm switch, EVQQ2 series http://www.ladyada.net/library/eagle
TP1 TP3 TP4 = adafruit:PINHD-1X1: Pin header 1x1 for 0.1" spacing
U1 = R1SE-0505-R:R1SE-0505-R; COPYRIGHT: Copyright (C) 2022 Ultra Librarian. All rights reserved.; MANUFACTURER_PART_NUMBER: R1SE-0505-R; MFR_NAME: Recom Power
U2 = MAX14483AAP:MAX14483AAP+; COPYRIGHT: Copyright (C) 2022 Ultra Librarian. All rights reserved.; MANUFACTURER_PART_NUMBER: MAX14483AAP+; MFR_NAME: Maxim Integrated Products
U3 U4 = ADP151AUJZ-3.3:ADP151AUJZ-3.3; COPYRIGHT: Copyright (C) 2022 Ultra Librarian. All rights reserved.; MANUFACTURER_PART_NUMBER: ADP151AUJZ-1.2-R7; MFR_NAME: Analog Devices Inc
U$2 U$5 U$6 = adafruit:FIDUCIAL: For use by pick and place machines to calibrate the vision/machine, 1mm

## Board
PCB Matrix Packages
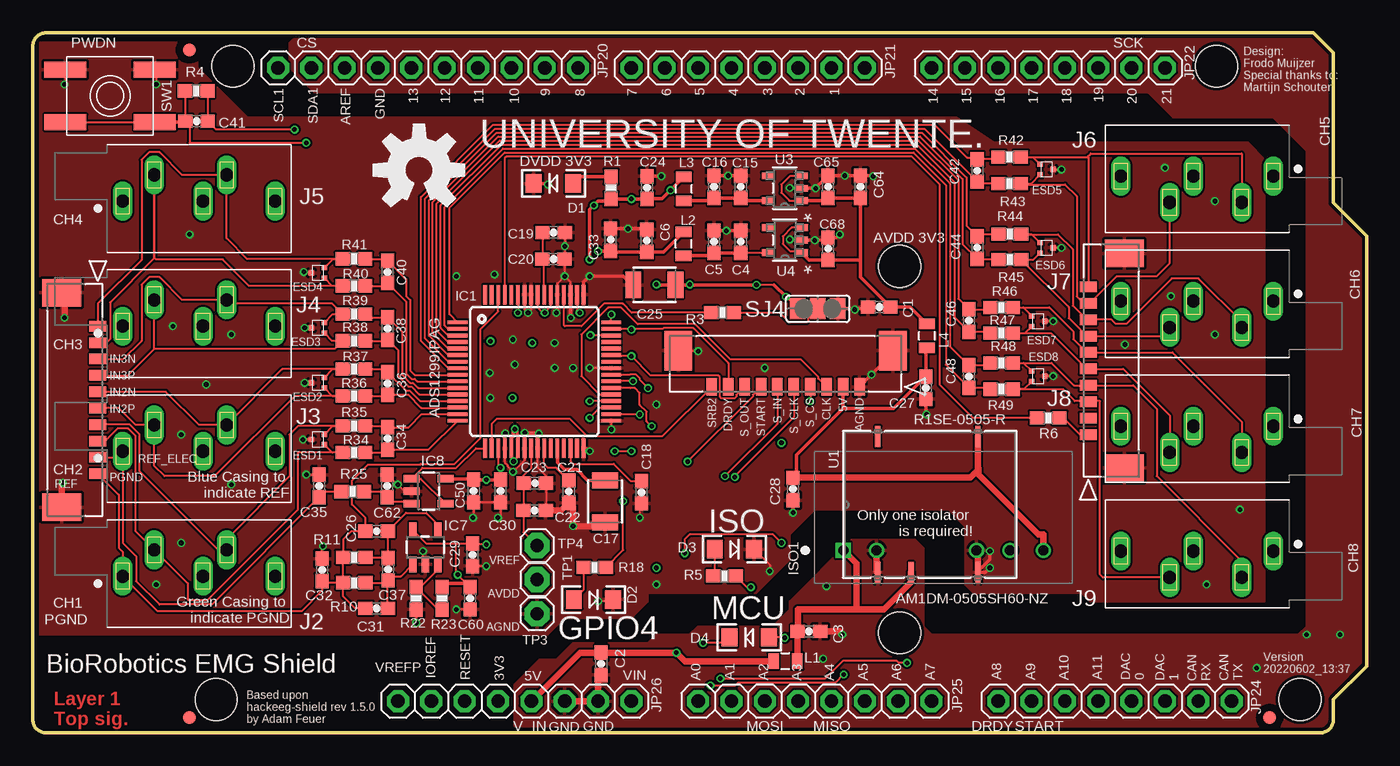
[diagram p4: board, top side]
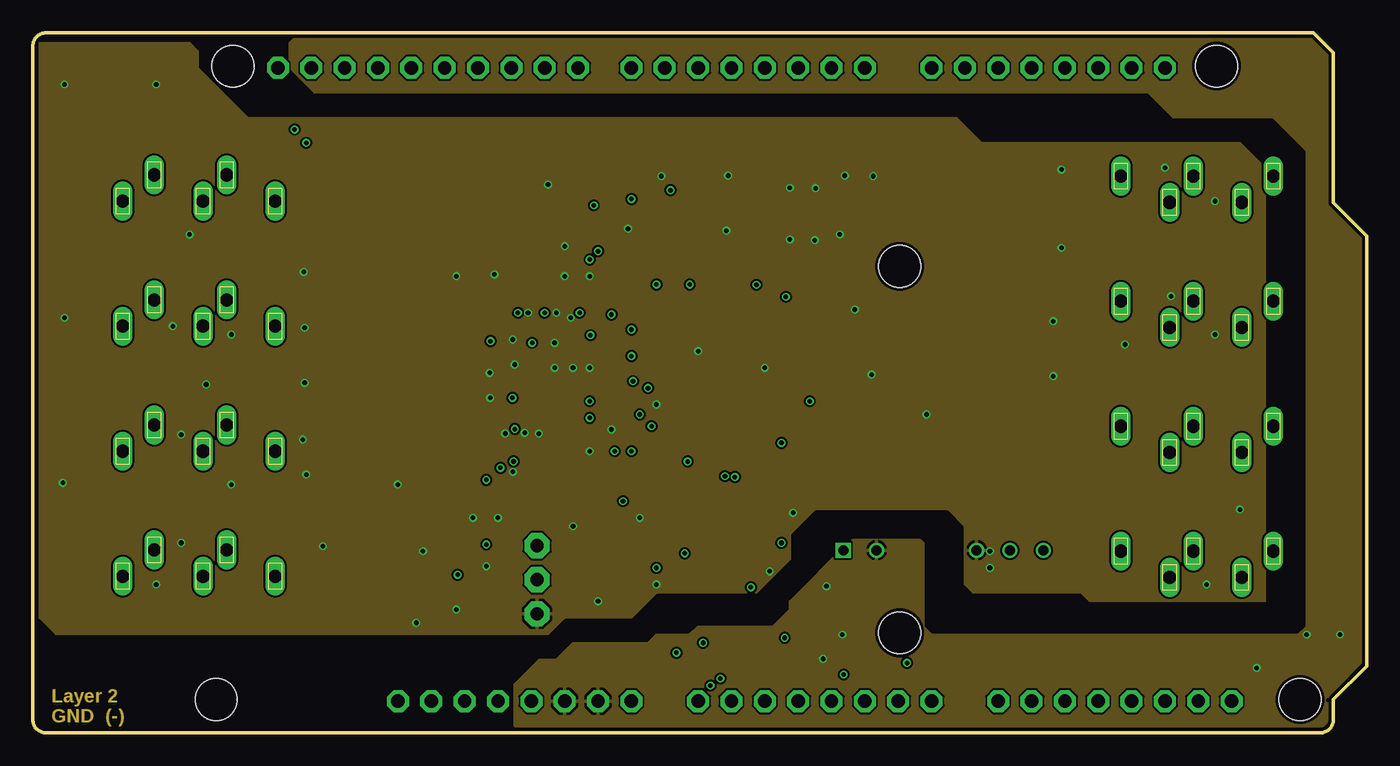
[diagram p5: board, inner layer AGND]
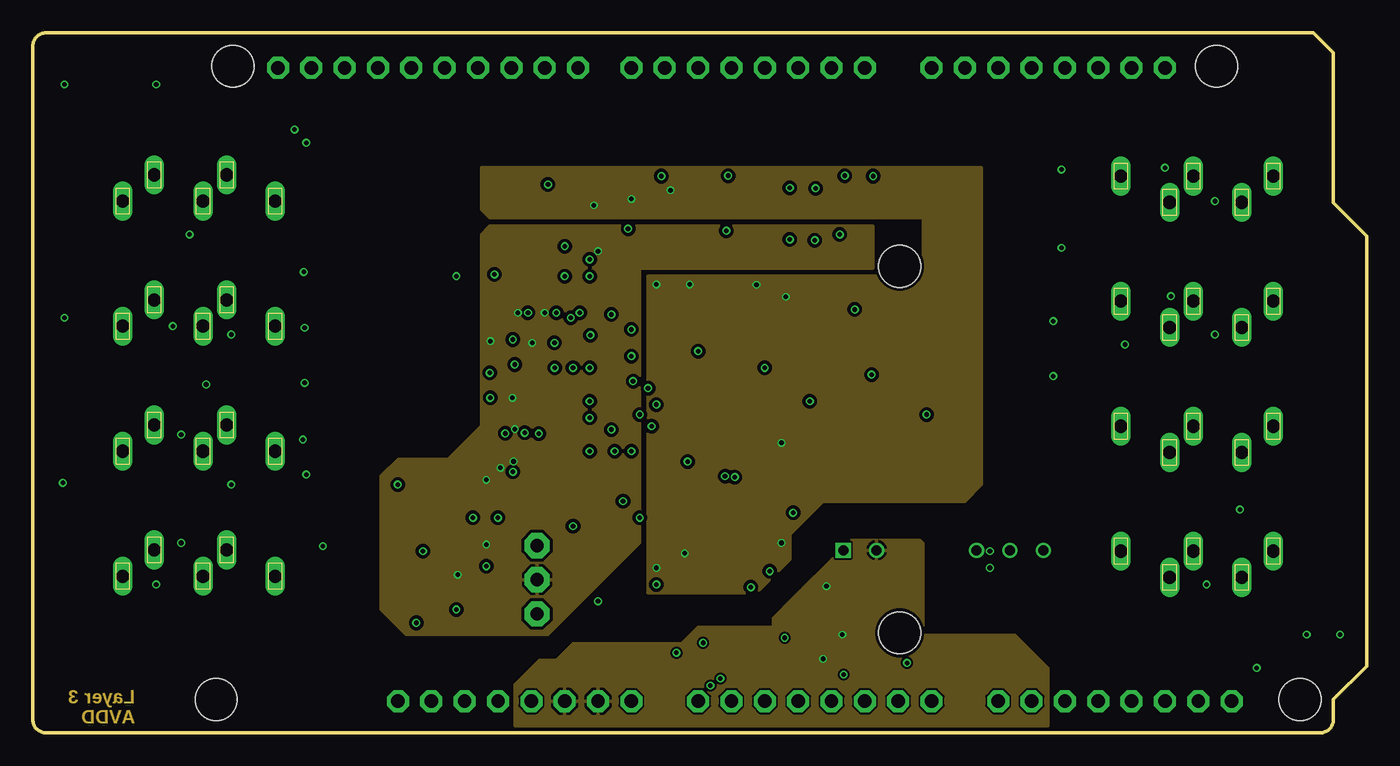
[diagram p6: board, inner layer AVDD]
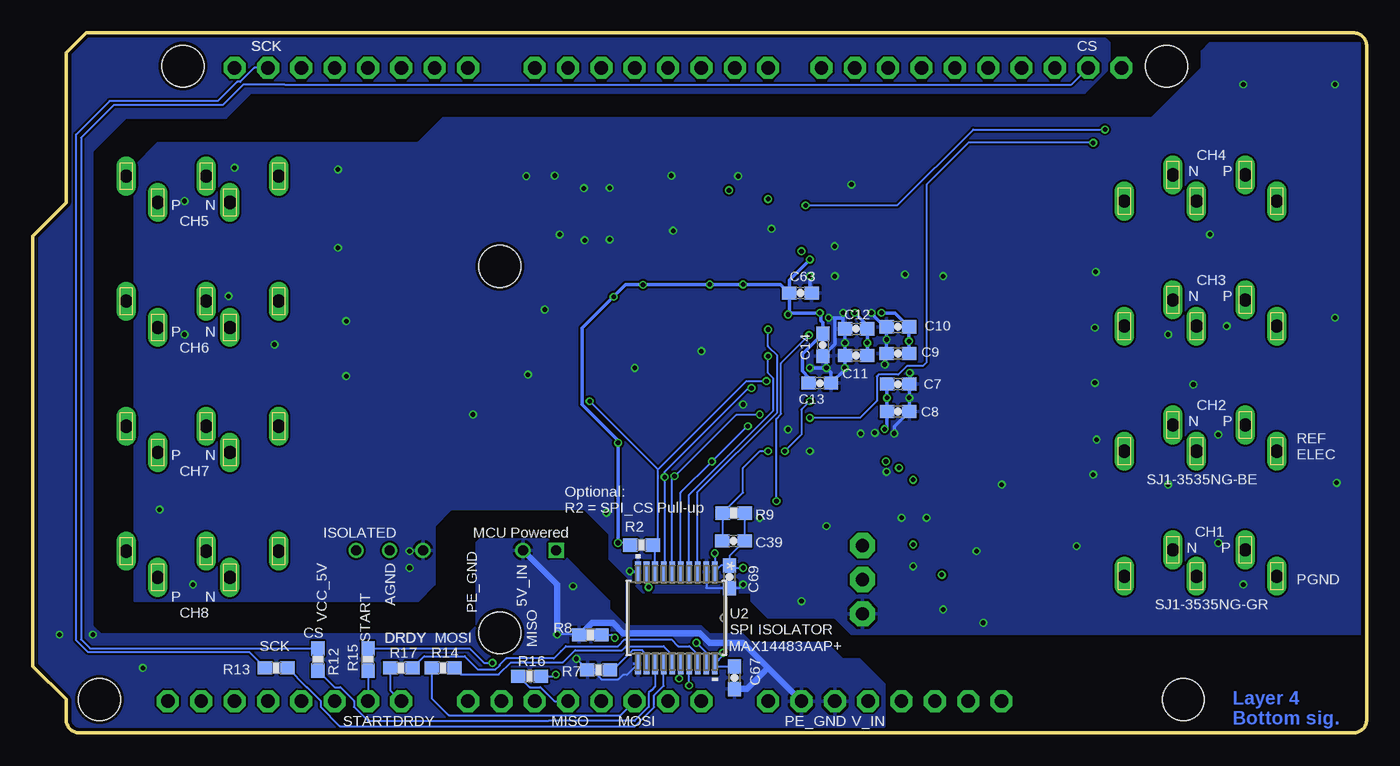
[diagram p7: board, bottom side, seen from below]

Size 101.6 x 53.34 mm. Coordinates in mm from the lower left corner, seen from the top.
Outline: 97.54,53.34 99.06,51.82 99.06,40.39 101.6,37.85 101.6,5.08 99.06,2.54 99.06,1 arc-90 98.06,0 1,0 arc-90 0,1 0,52.34 arc-90 1,53.34 97.54,53.34
Copper layers (1+2*15+16): Top 0.018mm / dielectric 0.36mm / AGND 0.035mm / dielectric 0.71mm / AVDD 0.035mm / dielectric 0.2mm / Bottom 0.018mm
Design rules "eC_4Layer_PClass6_BaseCopperO18-I35_eCDefault *": minimum track width 0.15mm, minimum drill 0.35mm, track to track 0.15mm, track to pad 0.15mm, pad to pad 0.15mm, via to via 0.15mm, smd to smd 0mil, copper to edge 0.25mm, drill to drill 0.35mm, minimum pad ring 0.175mm, minimum via ring 0.125mm, stop-mask expansion 0mil, vias tented up to drill 0.45mm, thermal gap 0.2mm
Holes 3.2 mm at 96.52,2.54 15.24,50.8 90.17,50.8 13.97,2.54 66.04,35.56 66.04,7.62

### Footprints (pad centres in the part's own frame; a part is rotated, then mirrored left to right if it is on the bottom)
0603-CAP = smd 1.1 x 1: 1 -0.85,0; 2 0.85,0
1210 = smd 1.2 x 2: 1 -1.6,0; 2 1.6,0
LED-1206 = smd 1.2 x 1.4: A -1.5,0; C 1.5,0
SOT-723 = smd 0.4 x 0.4: P$1 -0.4,-0.5; P$2 0.4,-0.5; P$3 0,0.5
TQFP64 = smd 1.5 x 0.285: 1 -5.85,3.75; 2 -5.85,3.25; 3 -5.85,2.75; 4 -5.85,2.25; 5 -5.85,1.75; 6 -5.85,1.25; 7 -5.85,0.75; 8 -5.85,0.25; 9 -5.85,-0.25; 10 -5.85,-0.75; 11 -5.85,-1.25; 12 -5.85,-1.75; 13 -5.85,-2.25; 14 -5.85,-2.75; 15 -5.85,-3.25; 16 -5.85,-3.75; 33 5.85,-3.75; 34 5.85,-3.25; 35 5.85,-2.75; 36 5.85,-2.25; 37 5.85,-1.75; 38 5.85,-1.25; 39 5.85,-0.75; 40 5.85,-0.25; 41 5.85,0.25; 42 5.85,0.75; 43 5.85,1.25; 44 5.85,1.75; 45 5.85,2.25; 46 5.85,2.75; 47 5.85,3.25; 48 5.85,3.75 | smd 0.285 x 1.5: 17 -3.75,-5.85; 18 -3.25,-5.85; 19 -2.75,-5.85; 20 -2.25,-5.85; 21 -1.75,-5.85; 22 -1.25,-5.85; 23 -0.75,-5.85; 24 -0.25,-5.85; 25 0.25,-5.85; 26 0.75,-5.85; 27 1.25,-5.85; 28 1.75,-5.85; 29 2.25,-5.85; 30 2.75,-5.85; 31 3.25,-5.85; 32 3.75,-5.85; 49 3.75,5.85; 50 3.25,5.85; 51 2.75,5.85; 52 2.25,5.85; 53 1.75,5.85; 54 1.25,5.85; 55 0.75,5.85; 56 0.25,5.85; 57 -0.25,5.85; 58 -0.75,5.85; 59 -1.25,5.85; 60 -1.75,5.85; 61 -2.25,5.85; 62 -2.75,5.85; 63 -3.25,5.85; 64 -3.75,5.85
SOT23-5 = smd 0.55 x 1.2: 1 -0.95,-1.3; 2 0,-1.3; 3 0.95,-1.3; 4 0.95,1.3; 5 -0.95,1.3
SIP1005W50P254L1965H1265Q7 = drill 0.76 pad 1.16 square: 1 -7.62,-2.495 | drill 0.76 pad 1.16: 2 -5.08,-2.495; 5 2.54,-2.495; 6 5.08,-2.495; 7 7.62,-2.495
CON_533981071 = smd 0.8 x 1.3: 1 0,0; 2 -1.25,0; 3 -2.5,0; 4 -3.75,0; 5 -5,0; 6 -6.25,0; 7 -7.5,0; 8 -8.75,0; 9 -10,0; 10 -11.25,0 | smd 2.1 x 3: 11 2.55,2.75; 12 -13.8,2.75
CUI_SJ1-3535N = drill 1 long: 1 0,0; 2 2.4,2; 3 7.9,2; 4 11.6,0; 5 6.1,0
1X10 = drill 1.016 pad 1.676 octagon: 1 -11.43,0; 2 -8.89,0; 3 -6.35,0; 4 -3.81,0; 5 -1.27,0; 6 1.27,0; 7 3.81,0; 8 6.35,0; 9 8.89,0; 10 11.43,0
1X08 = drill 1.016 pad 1.676 octagon: 1 -8.89,0; 2 -6.35,0; 3 -3.81,0; 4 -1.27,0; 5 1.27,0; 6 3.81,0; 7 6.35,0; 8 8.89,0
0805 = smd 0.8 x 1.2: 1 -0.9,0; 2 0.9,0
0603-RES = smd 1.1 x 1: 1 -0.85,0; 2 0.85,0
SJ_2 = smd 1.168 x 1.6: 1 -1.524,0; 2 0,0; 3 1.524,0
EVQ-Q2 = smd 3.2 x 1.2: A -3.4,-2; A' 3.4,-2; B -3.4,2; B' 3.4,2
1X01 = drill 1.016 pad 1.93 octagon: 1 0,0
R1SE-0505-R_RCP = smd 1.6 x 0.406: 1 -5.182,3.962; 2 -5.182,1.422; 4 -5.182,-3.658; 5 5.182,-3.658; 8 5.182,3.962
21-0056C_20_MXM = smd 1.613 x 0.432: 1 -3.499,2.925; 2 -3.499,2.275; 3 -3.499,1.625; 4 -3.499,0.975; 5 -3.499,0.325; 6 -3.499,-0.325; 7 -3.499,-0.975; 8 -3.499,-1.625; 9 -3.499,-2.275; 10 -3.499,-2.925; 11 3.499,-2.925; 12 3.499,-2.275; 13 3.499,-1.625; 14 3.499,-0.975; 15 3.499,-0.325; 16 3.499,0.325; 17 3.499,0.975; 18 3.499,1.625; 19 3.499,2.275; 20 3.499,2.925
UJ_5_ADI = smd 0.953 x 0.508: 1 -1.276,0.95; 2 -1.276,0; 3 -1.276,-0.95; 4 1.276,-0.95; 5 1.276,0.95
FIDUCIAL_1MM = smd 1 x 1: 1 0,0

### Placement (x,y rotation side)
C1  64.47,32.44 180 top
C2  43.29,5.26 270 top
C3  59.13,7.73 0 top
C4  53.92,37.41 90 top
C5  51.89,37.41 90 top
C6  46.76,37.49 90 top
C7  35.69,26.57 0 bottom
C8  35.69,24.49 0 bottom
C9  35.71,28.91 180 bottom
C10  35.71,30.94 180 bottom
C11  38.89,28.75 180 bottom
C12  38.89,30.78 180 bottom
C13  41.66,26.64 0 bottom
C14  41.43,29.57 270 bottom
C15  53.92,41.61 90 top
C16  51.89,41.61 90 top
C17  43.59,17.63 270 top
C18  46.35,18.34 270 top
C19  39.67,38.13 0 top
C20  39.65,36.09 0 top
C21  40.82,18.38 270 top
C22  38.22,16.94 0 top
C23  38.24,19.02 0 top
C24  46.79,41.55 90 top
C25  47.35,34.14 180 top
C26  26.19,15.37 0 top
C27  68.02,26.29 270 top
C28  57.89,18.57 270 top
C29  33.5,13.56 270 top
C30  35.62,18.43 90 top
C31  26.19,9.49 0 top
C32  22.03,12.42 270 top
C33  44.02,37.57 90 top
C34  27.03,22.43 90 top
C35  21.82,18.82 90 top
C36  27.03,26.62 90 top
C37  27.06,12.47 90 top
C38  27.03,30.81 90 top
C39  48.24,14.63 0 bottom
C40  27.03,35.13 90 top
C41  12.47,46.6 0 top
C42  71.93,42.85 270 top
C44  71.93,36.98 270 top
C46  71.3,31.42 270 top
C48  71.3,27.15 270 top
C50  33.58,18.43 270 top
C60  33.3,10.26 270 top
C62  26.98,18.82 90 top
C63  43.13,33.5 0 bottom
C64  63.04,41.61 90 top
C65  60.58,41.61 90 top
C67  48.15,4.19 270 bottom
C68  60.58,36.88 90 top
C69  48.53,11.89 270 bottom
D1  39.65,41.86 180 top
D2  42.7,10.16 0 top
D3  53.43,14 0 top
D4  54.57,7.28 180 top
ESD1  21.71,22.35 90 top
ESD2  21.71,26.67 90 top
ESD3  21.71,30.86 90 top
ESD4  21.71,35.05 90 top
ESD5  77.22,42.93 270 top
ESD6  77.22,36.96 270 top
ESD7  76.58,31.37 270 top
ESD8  76.58,27.18 270 top
IC1  38.2,27.53 0 top
IC7  29.9,14.15 0 top
IC8  30.15,18.42 270 top
ISO1  69.35,16.41 0 top
J1  62.97,26.37 0 top
J2  6.86,11.94 0 top
J3  6.86,21.46 0 top
J4  6.86,30.99 0 top
J5  6.86,40.51 0 top
J6  94.49,42.42 180 top
J7  94.49,32.89 180 top
J8  94.49,23.37 180 top
J9  94.49,13.84 180 top
J10  4.95,30.99 90 top
J11  80.39,22.73 270 top
JP20  30.1,50.67 0 top
JP21  54.48,50.67 0 top
JP22  77.34,50.67 0 top
JP24  82.42,2.41 0 top
JP25  59.56,2.41 0 top
JP26  36.7,2.41 0 top
L1  57.32,5.46 0 top
L2  49.56,37.26 90 top
L3  49.58,41.45 90 top
L4  68.1,30.25 90 top
R1  44.04,41.53 90 top
R2  55.23,14.31 0 bottom
R3  52.52,32.02 0 top
R4  12.44,48.91 0 top
R5  52.69,11.96 180 top
R6  77.34,24 180 top
R7  58.5,4.81 0 bottom
R8  59.14,7.48 0 bottom
R9  48.21,16.74 0 bottom
R10  24.49,11.44 180 top
R11  24.49,13.38 180 top
R12  79.88,5.59 270 bottom
R13  83.06,4.95 0 bottom
R14  70.36,4.95 0 bottom
R15  76.07,5.59 90 bottom
R16  63.75,4.32 0 bottom
R17  73.53,4.95 0 bottom
R18  42.8,12.62 180 top
R22  29.18,10.25 270 top
R23  31.17,10.25 270 top
R25  24.36,18.38 180 top
R34  24.46,21.36 0 top
R35  24.46,23.39 0 top
R36  24.46,25.68 0 top
R37  24.46,27.71 0 top
R38  24.46,29.87 0 top
R39  24.46,31.9 0 top
R40  24.46,34.06 0 top
R41  24.46,36.12 0 top
R42  74.4,43.87 180 top
R43  74.4,41.86 180 top
R44  74.42,38 180 top
R45  74.42,36.07 180 top
R46  73.79,32.41 180 top
R47  73.79,30.45 180 top
R48  73.79,28.19 180 top
R49  73.79,26.19 180 top
SJ4  59.79,32.31 0 top
SW1  5.88,48.54 0 top
TP1  38.4,11.67 0 top
TP3  38.4,9.07 0 top
TP4  38.4,14.26 0 top
U1  68.33,17.4 90 top
U2  52.58,8.76 270 bottom
U3  57.28,41.5 180 top
U4  57.29,37.54 180 top
U$1  [OSHW-LOGO-L]  29.41,42.88 0 top
U$2  11.91,1.17 0 top
U$5  11.91,52.04 0 top
U$6  94.21,1.17 0 top

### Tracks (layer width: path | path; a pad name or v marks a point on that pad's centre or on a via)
!PWDN  (via drill 0.35)
  Top 0.15: R4.1 11.59,46.57 11.55,46.53 | SW1.A 9.4,46.53 | v42.42,24 43.2,24.78 IC1.35 | C41.1 11.94,46.28 11.94,44.96 v20.83,44.96
  Top 0.254: C41.1 11.55,46.53 9.4,46.53 SW1.A'
  Bottom 0.15: v20.83,44.96 30.35,44.96 33.53,41.78 33.53,28.24 33.81,27.96 35.02,27.96 35.68,27.29 37.18,27.29 37.31,27.16 37.31,25.3 38.61,24 v42.42,24
!RESET  (via drill 0.35)
  Top 0.15: IC1.36 42.43,25.28 v42.42,25.27 | v44.32,21.46 v45.59,21.46
  Bottom 0.15: C39.1 49.09,16.72 R9.1 47.5,18.31 47.5,20.19 46.23,21.46 v45.59,21.46 | v42.42,25.27 43.05,24.64 43.05,22.73 v44.32,21.46
!SPI_CS  (via drill 0.35)
  Top 0.15: v45.72,26.8 44.06,26.8 IC1.39 | J1.4 59.21,25.31 v59.18,25.27
  Bottom 0.15: U2.8 54.2,14.13 R2.2 54,14.69 54,20.04 | v45.72,26.8 47.24,26.8 54,20.04 | v59.18,25.27 54,20.09 54,20.04
AGND  (via drill 0.35)
  Top 0.15: IC1.25 38.45,20.22 39.09,19.58 C23.2 39.09,16.96 C22.2 | SW1.B' 9.4,50.42 v9.4,49.4 | ESD4.P$3 20.7,35.05 v20.64,35.11 | ESD3.P$3 v20.7,30.86 | v20.7,30.86 | ESD2.P$3 v20.7,26.67 | v20.7,26.67 | C35.2 20.84,19.67 v20.83,19.69 | C62.2 27.73,18.92 v27.8,18.92 28.31,18.42 IC8.2 | v33.53,16.38 33.58,16.43 C50.2 C30.1 35.62,16.58 v35.43,16.38 | IC1.20 35.95,20.61 36.15,20.41 36.15,20.32 v36.57,19.89 37.45,20.77 IC1.23 | IC1.32 42.2,21.68 v42.42,21.46 | IC1.33 44.05,23.13 v44.07,23.11 | IC1.41 42.45,27.78 v42.42,27.81 | IC1.51 40.95,34.36 v40.51,34.8 | C20.2 40.51,36.08 | 40.51,36.08 v40.51,34.8 | IC1.53 39.95,34.24 v40.51,34.8 | IC1.58 37.45,32.27 v37.72,32 37.95,32.24 IC1.57 | C29.2 34.53,12.71 v34.54,12.7 | C60.2 33.29,9.4 v32.26,9.4 | v29.2,8.38 29.19,8.4 R22.2 | C32.1 22.03,14.16 v22.1,14.22 | D3.C 56.13,12.79 v56.13,12.32 | SW1.B 2.49,49.47 v2.41,49.4 | C19.2 40.52,37.34 | v40.52,37.08 40.52,36.09 40.51,36.08 | J1.11 65.52,29.08 | J1.12 50.64,29.12 v50.67,29.08 | D2.C 44.07,10.03 v43.05,10.03 | v77.72,27.18 | v77.72,27.18 ESD8.P$3 | ESD7.P$3 v77.72,31.37 | v77.72,31.37 | ESD6.P$3 v78.36,36.96 | v78.36,36.96 | ESD5.P$3 v78.36,42.93 | v78.36,42.93
  Top 0.152: IC7.2 29.72,13.02 v29.72,13.84 | C18.2 46.23,17.36 v46.23,16.38 | ESD1.P$3 v20.57,22.35 | v20.57,22.35
  Top 0.254: v72.9,13.84 72.9,13.21 71.98,12.29 U1.4 72.54,12.22 v72.9,12.57 | 65.52,29.08 65.52,28.92 v63.89,27.3 J1.1 | C28.2 57.89,16.78 v57.91,16.76 | IC1.20 35.95,22.78 v35.98,22.82 | IC1.23 37.45,22.85 v37.46,22.86 38.3,22.86 38.45,22.71 | IC1.25 38.45,22.71 | 38.45,22.71 v38.54,22.8 | IC1.53 39.95,32.08 v39.88,32 | IC1.51 40.95,31.65 v40.98,31.62 | IC1.49 41.95,34.33 v42.42,34.8 44.96,34.8 45.62,34.14 C25.2 | SJ4.3 62.55,32.31 | 62.55,32.31 v62.61,32.26 | J1.11 65.91,29.12 | 65.91,29.12 66.09,29.12 | C68.2 60.39,37.54 v59.56,37.54 U4.2 57.71,37.54 v57.66,37.59 | C68.2 60.83,37.98 | 65.53,29.51 65.91,29.12 | C5.2 v52.83,38.26 C4.2 | C1.2 63.49,32.31 62.55,32.31 | C27.2 68.02,24.31 v68.07,24.26 | C68.2 61.23,37.73 v61.47,37.97 | C33.2 v45.34,38.42 46.68,38.42 C6.2 | 40.52,37.34 v40.52,37.08 | C16.2 v52.96,42.45 C15.2 | v64.01,42.42 63.97,42.45 C64.2 v61.85,42.45 C65.2 v59.62,41.5 U3.2 57.69,41.5 v57.66,41.53 | C24.2 46.8,42.42 v47.88,42.42 | D1.C 39.17,41.86 v39.24,41.78
  Top 0.508: U1.4 71.98,13.82 ISO1.5 | C17.2 43.31,15.75 v41.15,15.75 41.15,17.21 C21.2 40.23,16.94 C22.2 | J10.11 2.41,33.33 v2.41,31.62 | J10.12 2.2,18.97 v2.29,19.05
  Bottom 0.15: U2.10 56.08,12.26 v56.13,12.32 | U2.2 50.3,11.06 50.29,11.04 C69.2 47.76,11.04 v47.5,11.3
  Bottom 0.254: v35.98,22.82 35.98,23.34 C8.2 v34.84,25.53 C7.2 34.8,26.61 v34.8,27.43 | v37.72,32 37.53,31.82 37.53,31.77 36.71,30.94 C10.2 v36.56,29.97 C9.2 36.7,28.77 v36.7,28.07 | v39.88,32 39.88,31.62 | 39.88,31.62 39.88,30.93 C12.2 v39.74,29.72 C11.2 39.74,27.83 v39.75,27.81 39.75,27.7 C13.2 40.81,27.47 v41.15,27.81 | v40.98,31.62 40.51,31.62 | 40.51,31.62 39.88,31.62 | 39.88,31.62 | v41.15,27.81 41.15,28.44 C14.2 40.51,29.63 40.51,31.62 | v42.42,27.81 v41.15,27.81 | v42.42,34.8 42.42,33.64 C63.2
  other vias: 86.69,33.27 91.95,17.02 35.16,34.92 32.26,34.8 11.94,37.97 11.3,22.73 15.11,18.92 11.3,14.48 9.4,11.3 13.21,26.54 15.11,30.35 10.67,30.99 55.75,27.81 86.23,43.05 90.04,40.51 90.04,30.35 83.19,29.59 89.41,11.3 47.5,25.02
  pour Top: 0.51,52.58 0.51,7.49 39.24,7.49 40.51,8.76 45.59,8.76 46.86,10.03 46.86,10.67 55.12,10.67 57.66,13.21 57.66,15.11 59.56,17.02 69.72,17.02 70.99,15.75 70.99,11.3 71.63,10.67 79.88,10.67 80.52,10.03 93.85,10.03 93.85,43.69 92.58,44.96 73.22,44.96 70.36,46.86 16.38,46.86 12.57,50.67 12.57,51.94 11.94,52.58
  pour Bottom: 0.51,52.58 0.51,7.49 39.24,7.49 40.51,8.76 45.59,8.76 46.86,10.03 46.86,10.67 55.12,10.67 57.66,13.21 57.66,15.11 59.56,17.02 69.72,17.02 70.99,15.75 70.99,11.3 72.26,10.03 93.85,10.03 93.85,43.18 92.08,44.96 72.26,44.96 70.36,46.86 16.38,46.86 12.57,50.67 12.57,51.94 11.94,52.58
  pour AGND: 0.51,52.58 11.94,52.58 12.57,51.94 12.57,50.67 16.38,46.86 70.36,46.86 72.26,44.96 91.95,44.96 93.85,43.05 93.85,10.03 80.52,10.03 79.88,10.67 71.63,10.67 70.99,11.3 70.99,15.75 69.72,17.02 59.56,17.02 57.66,15.11 57.66,13.21 55.12,10.67 47.5,10.67 45.59,8.76 40.51,8.76 39.24,7.49 1.78,7.49 0.51,8.76
AIN1N
  Top 0.152: R35.2 26.91,23.39 C34.2 28.61,23.28 29.62,24.28 IC1.15
AIN1P
  Top 0.152: R34.2 26.81,21.36 C34.1 30.15,21.58 IC1.16
AIN2N
  Top 0.152: R37.2 26.78,27.71 C36.2 28.42,26.07 28.71,26.07 29.5,25.28 IC1.13
AIN2P
  Top 0.152: R36.2 26.94,25.68 C36.1 28.59,25.77 29.59,24.77 32.33,24.77 IC1.14
AIN3N
  Top 0.152: R39.2 25.55,31.66 C38.2 28.12,30.57 28.12,27.3 28.74,26.68 28.96,26.68 29.35,26.29 IC1.11
AIN3P
  Top 0.152: R38.2 26.94,29.87 C38.1 27.81,29.17 27.81,27.18 28.62,26.37 28.84,26.37 29.43,25.78 IC1.12
AIN4N
  Top 0.152: R41.2 26.89,36.12 C40.2 28.45,34.56 28.45,33.28 28.75,32.98 28.75,27.61 29.08,27.28 IC1.9
AIN4P
  Top 0.152: R40.2 26.81,34.06 C40.1 28.45,32.86 28.45,27.4 28.87,26.98 29.09,26.98 29.28,26.78 IC1.10
AIN5N
  Top 0.152: R43.2 72.07,41.86 C42.2 67.9,46.03 35.19,46.03 29.86,40.7 29.86,30.06 31.64,28.28 IC1.7
AIN5P
  Top 0.152: R42.2 73.38,43.7 C42.1 71.79,43.85 71.15,43.85 68.66,46.34 35.07,46.34 29.56,40.83 29.56,29.86 31.64,27.78 IC1.8
AIN6N
  Top 0.152: IC1.5 31.64,29.28 30.47,30.46 30.47,40.45 35.44,45.43 67.58,45.43 70.82,42.19 70.82,37.25 C44.2 72,36.07 R45.2
AIN6P
  Top 0.152: R44.2 72.1,38 C44.1 71.12,38.64 71.12,42.32 67.71,45.73 35.32,45.73 30.17,40.58 30.17,30.26 31.64,28.78 IC1.6
AIN7N
  Top 0.152: R47.2 72.82,30.57 C46.2 70.18,31.69 70.18,41.97 67.33,44.82 35.69,44.82 31.07,40.2 31.07,30.85 31.64,30.28 IC1.3
AIN7P
  Top 0.152: R46.2 72.8,32.27 C46.1 70.48,33.08 70.48,42.1 67.46,45.12 35.57,45.12 30.77,40.33 30.77,30.65 31.64,29.78 IC1.4
AIN8N
  Top 0.152: R49.2 72.82,26.3 C48.2 69.55,28.05 69.55,41.75 67.08,44.22 35.94,44.22 31.73,40.01 31.73,31.9 IC1.1
AIN8P
  Top 0.152: R48.2 72.75,28 C48.1 69.85,29.45 69.85,41.88 67.21,44.52 35.82,44.52 31.38,40.08 31.38,31.05 31.64,30.78 IC1.2
AVDD  (via drill 0.35)
  Top 0.15: IC8.5 31.62,19.19 | C30.2 v35.62,20.19 35.45,20.37 IC1.19 | IC1.21 36.45,20.85 v36.62,20.68 36.95,21.01 IC1.22 | IC1.54 39.45,32.47 v38.99,32 38.86,32 38.45,32.41 IC1.56 | IC1.59 v36.95,32.01 v36.96,32 | 32.26,14.41 C29.1 34.48,14.41 v34.54,14.35
  Top 0.152: IC7.5 29.98,14.41 32.26,14.41 32.26,12.15 v32.36,12.04 | v32.36,12.04 33,11.41 C60.1 v32.36,12.04
  Top 0.254: IC1.21 36.45,22.47 36.56,22.58 36.56,22.99 v36.71,23.15 36.89,22.97 36.89,22.62 36.95,22.56 IC1.22 | L2.2 48.03,36.64 C6.1 44.09,36.64 C33.1 44,36.7 v43.05,36.7 | R23.1 31.48,11.41 33,11.41 | 31.45,19.28 IC8.5 33.49,19.37 C50.1 v34.54,19.28 C30.2
  Bottom 0.15: 34.86,29.72 v34.86,29.85 | 36.54,25.27 v36.54,25.53
  Bottom 0.254: 36.54,25.27 C8.1 36.54,23.33 v36.71,23.15 | v36.54,25.53 C7.1 | v36.96,32 35.93,32 C10.1 v34.86,29.85 | C9.1 34.86,29.72 | v38.99,32 38.04,31.05 C12.1 v38.04,29.72 C11.1
  pour AVDD (isolate 0.254): 34.8,38.61 34.16,37.97 34.16,23.37 31.62,20.83 27.81,20.83 26.54,19.56 26.54,9.4 28.45,7.49 39.24,7.49 46.23,14.48 46.23,35.43 64.01,35.43 64.01,38.61
BIASINV
  Top 0.15: IC1.61 35.94,33.39 35.94,43.79 36.07,43.92
  Top 0.152: 36.07,43.92 66.95,43.92 69.09,41.78 69.09,26.51 71.59,24 R6.2
CLK
  Top 0.15: J1.3 59.84,27 59.84,27.11 58.51,28.45 53.13,28.45 50.43,31.14 46.07,31.14 44.81,32.4 43.83,32.4 41.78,30.35 41.78,27.18 43.18,25.78 IC1.37
CLKSEL
  Top 0.15: R3.1 45.62,32.02 44.94,32.7 43.5,32.7 41.78,30.99 40.51,30.99 40.45,31.05 IC1.52
DRDY  (via drill 0.35)
  Top 0.15: v45.59,30.73 45.54,30.78 | 45.54,30.78 IC1.47 | 45.54,30.78 47.96,30.78 48.02,30.85 50.31,30.85 52.97,28.18 52.97,26.38 J1.9
  Bottom 0.15: U2.3 51,12.31 51,18.32 44.89,24.42 44.89,28.75 45.59,29.44 v45.59,30.73
DRDY_D69
  Bottom 0.152: R17.1 74.38,3.26 JP24.1
DVDD  (via drill 0.35)
  Top 0.15: IC1.48 44.05,31.86 v44.07,31.88 | IC1.50 41.45,32.21 v41.66,32 | R4.2 13.32,48.88 C41.2 13.96,45.97 v19.93,45.97 v19.94,45.97 | v57.02,14.48 56.39,15.11 50.04,15.11 49.66,14.73 v49.66,13.68 | 56.44,34.14 v55.12,34.14 | SJ4.1 v57.36,33.23
  Top 0.254: v47.5,34.16 47.52,34.14 C25.1 v55.12,34.14 | v57.36,33.23 56.44,34.14 | L3.2 v48.57,41.34 47.93,40.7 C24.1 46.76,40.68 v45.59,40.68 R1.1 43.88,40.51 43.05,40.51 v42.73,40.2 42.42,39.88 v42.42,36.07
  Bottom 0.15: R2.1 56.25,14.48 v57.02,14.48 | C69.1 49.17,12.74 U2.1 v49.66,13.68 | C69.1 48.36,12.57 v47.5,12.57 | R9.2 47.39,16.72 C39.2 48.53,13.49 C69.1 | v42.73,40.2 35.75,40.2 29.97,45.97 v19.94,45.97
  Bottom 0.254: 43.94,32 v41.66,32 41.55,31.9 41.55,31.38 41.43,31.26 C14.1 42.99,28.85 42.99,27.57 42.51,27.09 C13.1 | 43.94,32 v44.07,31.88 | C63.1 43.98,32.04 43.94,32 | C63.1 44.64,34.16 v47.5,34.16 v50.04,34.16 56.44,34.16 59.76,30.85 59.76,25.03 57.02,22.3 v57.02,22.1 v57.02,14.48 | v42.42,36.07 43.98,34.51 C63.1
  pour AVDD (isolate 0.254): 34.16,39.88 34.16,43.05 72.26,43.05 72.26,18.92 70.99,17.65 60.2,17.65 57.66,15.11 57.66,13.21 55.12,10.67 46.86,10.67 46.86,34.8 67.82,34.8 67.82,39.24 34.8,39.24
GPIO4  (via drill 0.35)
  Top 0.15: R18.1 44.96,13.93 v44.96,17.65 | v42.47,30.3 44.04,30.3 IC1.46
  Bottom 0.15: v44.96,17.65 44.96,23.94 44.59,24.3 44.59,28.18 v42.47,30.3
IN1N
  Top 0.15: J2.3 14.12,13.94 8.13,19.93 8.13,22.74 7.39,23.49 J10.7
  Top 0.152: ESD1.P$2 22.86,23.39 R35.1 23.59,23.37 20.19,23.37 19.56,22.73 19.56,19.56 14.76,14.76 J2.3
IN1P
  Top 0.15: J2.2 7.83,15.36 7.83,22.62 7.26,23.19 6.45,23.19 5.5,22.24 J10.8
  Top 0.152: ESD1.P$1 22.8,21.36 R34.1 20.18,21.36 20.18,17 13.29,10.11 11.8,10.11 11.8,11.4 J2.2
IN2N
  Top 0.15: J3.3 12.66,23.46 10.13,25.99 J10.5
  Top 0.152: ESD2.P$2 22.86,27.71 R37.1 19.01,27.71 J3.3
IN2P
  Top 0.15: J3.2 7.83,23.46 6.55,24.75 4.96,24.75 J10.6
  Top 0.152: ESD2.P$1 22.8,25.68 R36.1 19.96,25.68 13.84,19.56 10.03,19.56 9.26,20.33 J3.2
IN3N
  Top 0.15: J4.3 11.39,32.99 9.66,34.71 8.85,34.71 8.28,34.14 8.28,29.87 6.86,28.45 4.99,28.45 J10.3
  Top 0.152: ESD3.P$2 22.86,31.9 R39.1 22.8,32.71 15.03,32.71 J4.3
IN3P
  Top 0.15: J10.4 7.23,27.24 9.26,29.26
  Top 0.152: ESD3.P$1 22.8,29.87 R38.1 23,29.26 9.26,29.26 J4.2
IN4N
  Top 0.15: J10.1 4.95,32.71 8.28,36.04 8.28,43.67 8.85,44.24 9.66,44.24 11.39,42.51 J5.3
  Top 0.152: ESD4.P$2 22.88,36.12 R41.1 16.33,36.12 14.76,37.69 J5.3
IN4P
  Top 0.15: J5.2 9.26,36.18 5.88,32.8 5.88,30.01 5.59,29.72 4.97,29.72 J10.2
  Top 0.152: ESD4.P$1 22.8,34.06 R40.1 16.48,34.06 14.48,36.07 9.4,36.07 9.26,36.21 J5.2
IN5N
  Top 0.152: J6.3 86.59,35.79 85.6,34.8 82.58,34.8 80.51,32.73 J11.9 80.04,32.73 79.52,33.26 79.52,40.88 78.61,41.78 75.32,41.78 R43.1 76.05,41.86 ESD5.P$2
IN5P
  Top 0.152: R42.1 76.18,43.87 ESD5.P$1 | R42.1 80.39,43.87 J11.10 | R42.1 80.3,43.87 80.58,44.14 92.09,44.14 J6.2
IN6N
  Top 0.152: ESD6.P$2 76.23,36.07 R45.1 78.91,32.43 78.91,31.59 80.27,30.23 J11.7 85.93,30.23 J7.3
IN6P
  Top 0.152: ESD6.P$1 76.08,38 R44.1 75.3,37.97 78.09,37.97 79.21,36.85 79.21,32.54 80.27,31.48 J11.8 82.17,31.48 82.48,31.17 83.29,31.17 86.75,34.62 88.79,34.62 92.09,31.32 J7.2
IN7N
  Top 0.152: ESD7.P$2 75.57,30.46 R47.1 77.55,30.46 80.27,27.73 J11.5 83.05,27.73 86.59,24.2 J8.3
IN7P
  Top 0.152: ESD7.P$1 75.44,32.41 R46.1 77.43,32.41 79.25,30.59 79.25,30.01 80.27,28.98 J11.6 80.52,28.98 86.81,28.98 92.09,23.7 J8.2
IN8N
  Top 0.152: ESD8.P$2 75.49,26.19 R49.1 78.45,26.19 79.36,25.27 80.35,25.27 J11.3 80.43,25.27 81.28,25.27 81.28,12.07 81.51,11.84 J9.3
IN8P
  Top 0.152: ESD8.P$1 75.47,28.19 R48.1 77.6,28.19 79.31,26.48 J11.4 83.81,26.48 85.6,24.69 85.6,19.56 92.09,13.07 J9.2
N$1
  Top 0.15: 53.95,36.59 U4.5
  Top 0.152: 53.95,36.59 C4.1
  Top 0.254: C4.1 C5.1 51.69,36.36 L2.1
N$2
  Top 0.254: U3.5 54.13,40.55 C15.1 C16.1 51.69,40.55 L3.1
N$3
  Top 0.254: C17.1 42.27,19.23 41.44,20.06 40.5,20.06 39.95,20.61 IC1.28
N$4
  Top 0.152: IC1.30 40.95,20.69 41.15,20.5 44.24,20.5 45.54,19.19 C18.1
N$5
  Top 0.152: C19.1 38.82,36.12 C20.1 38.95,35.94 IC1.55
N$6
  Top 0.508: L1.2 58.22,7.68 C3.1 58.27,9.4 62.74,9.4 | U1.2 66.9,11.46 64.84,9.4 62.74,9.4 | 62.74,9.4 62.74,12.9 ISO1.1
N$7  (via drill 0.35)
  Top 0.15: v57.27,7.24 57.24,7.28 D4.A
  Bottom 0.15: R8.2 57.52,7.48 v57.27,7.24
N$8
  Top 0.152: C21.1 39.86,20.19 39.24,20.19 38.95,20.48 IC1.26
N$9
  Top 0.15: D3.A 51.93,12.05 R5.2
N$10
  Top 0.152: R6.1 78.49,24 79.76,22.73 J11.1
N$11  (via drill 0.35)
  Top 0.15: v54.69,11.09 54.4,11.09 R5.1
  Bottom 0.15: U2.9 54.85,11.25 v54.69,11.09
N$12
  Bottom 0.15: 67.67,4.81 66.37,4.81 66.06,5.12 66.06,5.17 65.55,5.68 61.92,5.68 61.37,6.22
  Bottom 0.152: U2.18 50.91,5.31 50.91,5.91 51.6,6.6 52.45,6.6 52.96,7.11 56.52,7.11 57.03,6.6 60.99,6.6 61.37,6.22 | R17.2 71.79,5.84 68.71,5.84 67.82,4.95 67.67,4.81
N$13  (via drill 0.35)
  Top 0.15: D4.C 52.65,6.86 v51.05,6.86
  Bottom 0.15: v51.05,6.86 50.3,6.11
  Bottom 0.152: 50.3,6.11 U2.19
N$14
  Top 0.15: R18.2 41.95,10.91 D2.A
N$15
  Top 0.15: R23.2 30.89,9.4 R22.1 29.51,11.1 30.85,12.43 IC7.3
N$16
  Bottom 0.15: U2.13 54.2,3.53 | 54.48,3.25 54.69,3.05 54.69,1.97 55.75,0.91 62.33,0.91
  Bottom 0.152: R12.2 78.62,3.48 78.17,3.48 77.14,2.44 77.14,1.97 76.07,0.91 62.33,0.91 | 54.2,3.53 54.48,3.25
N$17
  Bottom 0.15: R13.2 80.73,3.48 80.71,3.48 79.68,2.44 79.68,1.97 78.21,0.51 55.73,0.51 54.28,1.96 54.28,2.85 53.55,3.58 U2.14
N$18
  Top 0.152: R10.1 26.88,11.44 C37.1 | C31.2 27.04,11.6 C37.1 | C37.1 27.38,11.94 28.04,11.94 IC7.1
N$19
  Top 0.254: D1.A 41.67,42.38 R1.2
N$20
  Top 0.15: R3.2 56.86,32.02 57.59,31.29 58.95,31.29 59.08,31.42 59.08,31.6 SJ4.2
N$21
  Bottom 0.15: 66.11,4.45 65.18,5.37 61.21,5.37
  Bottom 0.152: R14.2 69,4.45 66.11,4.45 | 61.21,5.37 60.29,6.3 56.72,6.3 56.41,6.6 53.55,6.6 52.9,5.96 U2.15
N$22  (via drill 0.35)
  Top 0.15: 60.71,4.49 60.35,4.13 v52.37,4.13
  Top 0.152: v66.59,5.33 65.95,5.33 65.81,5.48 61.7,5.48 60.71,4.49
  Bottom 0.15: v52.37,4.13 52.37,5.14 U2.16
  Bottom 0.152: R15.2 68.33,6.44 67.22,5.33 v66.59,5.33
N$23  (via drill 0.35)
  Top 0.152: v61.76,4.45 61.13,3.81 53.72,3.81 53.52,3.61 v51.61,3.61
  Bottom 0.152: v51.61,3.61 51.61,4.75 51.6,4.75 U2.17 | R16.2 61.89,4.32 v61.76,4.45
N$26
  cutout AVDD: 98.6,2.59 98.58,2.49 arc180
N$44
  Bottom 0.152: U2.12 54.85,5.96 55.19,6.3 55.91,6.3 57.4,4.81 R7.2
N$54
  Top 0.152: R11.1 27,13.38 C37.2 27.04,13.34 C26.2 28.43,16.76 29.97,16.76 30.85,15.89 IC7.4
N$55
  cutout AGND: 98.63,2.57 98.6,2.46 arc180
PE  (via drill 0.35)
  Top 0.508: U1.1 64.27,12.31 ISO1.2 | JP26.6 JP26.7 43.05,4.17 C2.2 | C3.2 61.43,7.73 v61.66,7.49
  Bottom 0.15: R8.1 60,7.49 v61.66,7.49 | 57.02,4.08 56.97,4.08 56.64,4.41
  Bottom 0.152: 59.56,4.6 R7.1 | 57.01,4.08 57.02,4.08 58.3,4.08 59.02,4.81 R7.1 | 55.83,5.26 U2.11 56.35,4.41 56.64,4.41 | R7.1 v60.2,5.64
  Bottom 0.508: ISO1.2 61.66,11.3 v61.66,7.49 | R8.1 59.91,7.48 59,8.38 57.42,8.38 56.63,7.59 50.79,7.59 50.06,6.86 47.5,6.86 45.59,4.95 | 43.18,2.41 JP26.7 45.59,4.95 | C67.2 47.2,3.34 45.59,4.95
  other vias: 93.22,4.95 99.57,7.49 97.03,7.49 60.45,11.18
  pour AVDD: 36.7,0.51 36.7,3.68 38.61,5.59 39.88,5.59 41.15,6.86 49.4,6.86 50.67,8.13 56.39,8.13 56.39,8.76 62.36,14.73 67.56,14.73 67.82,14.48 67.82,7.49 74.8,7.49 77.34,4.95 77.34,0.51 76.71,-0.13 37.34,-0.13
  pour Bottom: 36.7,2.41 36.7,3.68 38.61,5.59 39.88,5.59 41.15,6.86 46.86,6.86 47.5,7.49 48.13,7.49 50.04,7.49 50.67,8.13 53.85,8.13 56.39,8.13 57.02,8.76 57.66,9.4 57.66,10.03 62.36,14.73 65.41,14.73 67.56,14.73 67.82,14.48 67.82,8.13 68.45,7.49 86.87,7.49 96.39,7.49 97.03,8.13 97.03,44.32 95.12,46.23 94.49,46.86 88.14,46.86 86.87,46.86 84.96,48.77 84.33,48.77 21.46,48.77 19.56,50.67 19.56,52.58 20.19,53.21 69.72,53.21 97.66,53.21 98.93,51.94 98.93,40.51 101.47,37.97 101.47,5.59 98.93,3.05 98.93,1.14 98.3,0.51 97.66,-0.13 49.4,-0.13 37.34,-0.13 36.7,0.51
  pour Top: 38.61,5.59 39.88,5.59 41.15,6.86 46.86,6.86 47.5,7.49 50.04,7.49 50.67,8.13 56.39,8.13 57.02,8.76 57.66,9.4 57.66,10.03 62.36,14.73 67.18,14.73 67.82,14.1 67.82,13.21 67.82,8.13 68.45,7.49 72.9,7.49 96.39,7.49 97.03,8.13 97.03,44.32 94.49,46.86 86.87,46.86 84.96,48.77 69.72,48.77 21.46,48.77 19.56,50.67 19.56,52.58 20.19,53.21 75.44,53.21 97.66,53.21 98.93,51.94 98.93,40.51 101.47,37.97 101.47,5.59 98.93,3.05 98.93,1.14 97.66,-0.13 37.34,-0.13 36.7,0.51 36.7,3.68
  pour AGND: 36.7,0.51 36.7,3.68 38.61,5.59 39.88,5.59 41.15,6.86 46.86,6.86 47.5,7.49 50.04,7.49 50.67,8.13 56.39,8.13 57.66,9.4 57.66,10.03 62.1,14.48 62.23,14.6 62.36,14.6 62.48,14.73 67.56,14.73 67.82,14.48 67.82,8.13 68.45,7.49 88.14,7.49 96.39,7.49 97.03,8.13 97.03,44.32 94.49,46.86 86.87,46.86 84.96,48.77 84.33,48.77 21.46,48.77 19.56,50.67 19.56,52.58 20.19,53.21 71.63,53.21 97.66,53.21 98.93,51.94 98.93,40.51 101.47,37.97 101.47,5.59 98.93,3.05 98.93,1.14 97.66,-0.13 53.85,-0.13 37.34,-0.13
PGND
  Top 0.15: J10.10 6.56,18.13 6.56,14.08 6.86,13.79 J2.1
  Top 0.152: R10.2 R11.2 23.64,14.75 24.26,15.37 C26.1 25.34,16.38 24.31,17.41 24.31,19.23 25.53,20.45 29.5,20.45 29.55,20.5 32.13,20.5 34.08,22.45 34.08,30.75 35.45,32.11 IC1.62 | C31.1 24.54,9.49 23.64,10.4 R10.2 | R10.2 22.16,11.44 C32.2 22.03,10.84 20.46,9.27 9.52,9.27 J2.1
REF_ELEC
  Top 0.152: R25.1 26.57,18.38 C62.1 27.3,17.65 28.66,17.65 IC8.3
REF_ELEC_CON
  Top 0.15: C35.1 13.66,9.81 11.26,9.81 9.65,9.78 7.87,11.56 7.87,13.46 6.86,14.48 J3.1 6.38,20.99 J10.9
  Top 0.152: C35.1 22.23,18.38 R25.2
SPI2_CS
  Bottom 0.15: 82.42,49.4 85.58,49.4 87.15,47.83 95.42,47.83 97.92,45.34 97.92,7.11 97.24,6.44 R12.1
  Bottom 0.152: JP20.2 22.48,49.4 82.42,49.4
SPI2_MISO
  Bottom 0.15: R16.1 63.76,3.48 62.93,3.48 61.87,2.41 JP25.5
SPI2_MOSI
  Bottom 0.15: R14.1 71.21,2.63 69.93,1.35 56.82,1.35 JP25.3
SPI2_SCK
  Bottom 0.15: JP22.7 84.73,50.67 85.79,49.61 86.03,49.61 87.5,48.13 95.76,48.13 98.3,45.59 98.3,7.07 97.37,6.14 85.09,6.14 R13.1
SPI_CLK  (via drill 0.35)
  Top 0.15: v46.86,26.27 46.24,26.89 46.24,27.01 45.94,27.32 45.5,27.32 45.46,27.28 IC1.40 | J1.5 57.96,24.06 53.47,19.57 v53.47,19.5
  Bottom 0.15: U2.7 53.47,12.34 v53.47,19.5 53.47,19.89 47.09,26.27 v46.86,26.27
SPI_IN  (via drill 0.35)
  Top 0.15: v46.23,24.26 44.08,24.26 IC1.34 | J1.6 56.71,23.55 v52.72,19.56
  Bottom 0.15: U2.6 52.9,19.36 | 52.9,19.36 48.01,24.26 v46.23,24.26 | v52.72,19.56 52.9,19.38 52.9,19.36
SPI_OUT  (via drill 0.35)
  Top 0.15: IC1.43 44.13,28.7 v45.59,28.7 47.05,27.25 52.21,27.25 52.34,27.11 52.34,25.63 52.47,25.5 53.46,25.5 53.59,25.63 53.59,25.75 J1.8
  Bottom 0.15: U2.4 51.6,18.14 45.2,24.55 45.2,27.01 45.59,27.41 v45.59,28.7
SRB1
  Top 0.152: IC8.4 29.55,19.37 IC8.1 29.68,20.19 32.26,20.19 33.75,21.68 IC1.17
SRB2
  Top 0.15: IC1.18 34.96,23.54 35.34,23.93 40.92,23.93 42.26,22.59 47.93,22.59 J1.10
START  (via drill 0.35)
  Top 0.15: v47.13,23.37 46.75,23.73 46.75,24.47 46.23,25 46.23,25.91 45.86,26.27 45.5,26.27 45.49,26.28 IC1.38 | J1.7 54.84,25.75 54.84,25.63 54.71,25.5 v49.88,20.67
  Bottom 0.15: U2.5 52.25,18.31 v49.88,20.67 47.16,23.37 v47.13,23.37
START_D68
  Bottom 0.152: R15.1 JP24.2
VCC_5V
  Top 0.254: C28.1 58.03,19.56 58.17,19.56 58.17,21.16 61.71,24.71 | J1.2 61.71,24.71 | C27.1 68.02,27.18 | 68.02,27.18 68.02,29.28 L4.1 | 61.71,24.71 65.55,24.71 68.02,27.18
  Top 0.508: ISO1.7 76.97,15.11 76.58,15.11 72.01,19.69 71.98,20.8 U1.5 71.98,20.04 71.41,19.47 57.94,19.47 C28.1
VCC_5V_FILTERED
  Top 0.15: U4.3 57.8,38.49 57.13,37.83 57.13,37.25 57.67,36.71 | U3.3 58.52,42.42 57.66,42.42 57.02,41.78 57.02,41.15 57.62,40.55 U3.1
  Top 0.152: 57.67,36.71 58.45,36.71 U4.1
  Top 0.254: L4.2 66.81,32.44 C1.1 63.04,34.72 63.04,35.99 | 63.04,35.99 63,36.03 C68.1 59.13,36.03 U4.1 | 63.04,35.99 C64.1 C65.1 60.37,40.55 U3.1
VCC_MCU  (via drill 0.35)
  Top 0.508: JP26.5 41.67,6.11 C2.1 v49.02,6.11 49.67,5.46 L1.1
  Bottom 0.15: U2.20 49.02,5.9 v49.02,6.11
  Bottom 0.152: C67.1 49.43,5.04 U2.20
VREFP
  Top 0.15: IC1.24 37.97,21.66 37.97,20.19 37.39,19.61 C23.1 37.39,16.96 C22.1 37.37,15.3 TP4.1

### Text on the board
Top: Layer 1 / Top sig.
AGND: Layer 2 / GND (-)
AVDD: Layer 3 / AVDD
Bottom: Layer 4 / Bottom sig.
tPlace: SCL1 | SDA1 | AREF | GND | 13 | 12 | 11 | 10 | 9 | 8 | 7 | 6 | 5 | 4 | 3 | 2 | 1 | 14 | 15 | 16 | 17 | 18 | 19 | 20 | 21 | VREFP | 5V | VIN | IOREF | RESET | 3V3 | A0 | A1 | A2 | A3 | A4 | A5 | A6 | A7 | A8 | A9 | A10 | A11 | DAC / 0 | DAC / 1 | CAN / RX | CAN / TX | GND | GND
tNames: PWDN | CS | SCK | Design: / Frodo Muijzer / Special thanks to: / Martijn Schouten | UNIVERSITY OF TWENTE. | CH5 | DVDD 3V3 | U3 | CH4 | AVDD 3V3 | U4 | CH6 | CH3 | IN3N | IN3P | IN2N | SRB2 / DRDY / S_OUT / START / S_IN / S_CLK / S_CS / CLK / 5V / AGND | IN2P | ADS1299IPAG | CH7 | U1 | REF_ELEC | CH2 | Blue Casing to / indicate REF | REF | PGND | ISO | Only one isolator / is required! | VREF | CH8 | Green Casing to / indicate PGND | AVDD | AM1DM-0505SH60-NZ | CH1 | AGND | MCU | PGND | GPIO4 | BioRobotics EMG Shield | Version / 20220602_13:37 | Based upon / hackeeg-shield rev 1.5.0 / by Adam Feuer | V_IN | MOSI | MISO | DRDY | START
bNames: CS | SCK | SCK | CH4 / N P | P N / CH5 | CH3 / N P | P N / CH6 | CH2 / N P | REF / ELEC | P N / CH7 | SJ1-3535NG-BE | Optional: / R2 = SPI_CS Pull-up | MCU Powered | ISOLATED | CH1 / N P | PE_GND | 5V_IN | AGND | VCC_5V | PGND | START | SJ1-3535NG-GR | MISO | P N / CH8 | U2 / SPI ISOLATOR | MOSI | DRDY | DRDY | CS | SCK | V_IN | PE_GND | MOSI | MISO | DRDY | START

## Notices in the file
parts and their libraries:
SparkFun-Passives: Licensing: CC v3.0 Share-Alike You are welcome to use this library for commercial purposes.
